(* Logix 5000 AddOnInstructionDefinition export HI6200_Faceplate_IT_AOI; software revision 30.00 *)

ADD_ON_INSTRUCTION HI6200_Faceplate_IT_AOI   (* revision 1.1, vendor Hardy Process Solutions *)
// HMI AOI for the Integrated Technician data.
VAR_IN_OUT
   Inp_hi6200 : _0102:Hardy6200Series_F6857DC7:I:0; {required}
   Out_hi6200 : _0102:Hardy6200Series_52E4DDE0:O:0; {required}
END_VAR
VAR_INPUT
   IT_Status : DINT;   // Integrated Technician status indication
   pm_4990 : REAL;   // WT ch 0
   pm_4991 : REAL;   // Wt ch 1
   pm_4992 : REAL;   // WT ch 2
   pm_4993 : REAL;   // WT ch 3
   pm_4994 : REAL;   // WT ch 4
   pm_4995 : REAL;   // WT ch 5
   pm_4996 : REAL;   // WT ch 6
   pm_4997 : REAL;   // WT ch 7
   pm_49A0 : REAL;   // mv/v ch 0
   pm_49A1 : REAL;   // mv/v ch 1
   pm_49A2 : REAL;   // mv/v ch 2
   pm_49A3 : REAL;   // mv/v ch 3
   pm_49A8 : REAL;   // mv/v ref 1
   pm_49A4 : REAL;   // mv/v ch 4
   pm_49A5 : REAL;   // mv/v ch 5
   pm_49A6 : REAL;   // mv/v ch 6
   pm_49A7 : REAL;   // mv/v ch 7
   pm_49A9 : REAL;   // mv/v ref 2
   pm_49B0 : REAL;   // RAW VAR ch 0
   pm_49B1 : REAL;   // RAW VAR ch 1
   pm_49B2 : REAL;   // RAW VAR ch 2
   pm_49B3 : REAL;   // RAW VAR ch 3
   pm_49B8 : REAL;   // RAW VAR ref 1
   pm_49B4 : REAL;   // RAW VAR ch 4
   pm_49B5 : REAL;   // RAW VAR ch 5
   pm_49B6 : REAL;   // RAW VAR ch 6
   pm_49B7 : REAL;   // RAW VAR ch 7
   pm_49B9 : REAL;   // RAW VAR ref 2
   pm_49C0 : REAL;   // WAVERSAVER VAR ch 0
   pm_49C1 : REAL;   // WAVERSAVER VAR ch 1
   pm_49C2 : REAL;   // WAVERSAVER VAR ch 2
   pm_49C3 : REAL;   // WAVERSAVER VAR ch 3
   pm_49C8 : REAL;   // WAVERSAVER VAR ref 1
   pm_49C4 : REAL;   // WAVERSAVER VAR ch 4
   pm_49C5 : REAL;   // WAVERSAVER VAR ch 5
   pm_49C6 : REAL;   // WAVERSAVER VAR ch 6
   pm_49C7 : REAL;   // WAVERSAVER VAR ch 7
   pm_49C9 : REAL;   // WAVERSAVER VAR ref 2
   pm_49D0 : DINT;   // RAW VAR results ch 0
   pm_49D1 : DINT;   // RAW VAR results ch 1
   pm_49D2 : DINT;   // RAW VAR results ch 2
   pm_49D3 : DINT;   // RAW VAR results ch 3
   pm_49D8 : DINT;   // RAW VAR results ref 1
   pm_49D4 : DINT;   // RAW VAR results ch 4
   pm_49D5 : DINT;   // RAW VAR results ch 5
   pm_49D6 : DINT;   // RAW VAR results ch 6
   pm_49D7 : DINT;   // RAW VAR results ch 7
   pm_49D9 : DINT;   // RAW VAR results ref 2
   pm_49E0 : DINT;   // WAVERSAVER VAR results ch 0
   pm_49E1 : DINT;   // WAVERSAVER VAR results ch 1
   pm_49E2 : DINT;   // WAVERSAVER VAR results ch 2
   pm_49E3 : DINT;   // WAVERSAVER VAR results ch 3
   pm_49E8 : DINT;   // WAVERSAVER VAR results ref 1
   pm_49E4 : DINT;   // WAVERSAVER VAR results ch 4
   pm_49E5 : DINT;   // WAVERSAVER VAR results ch 5
   pm_49E6 : DINT;   // WAVERSAVER VAR results ch 6
   pm_49E7 : DINT;   // WAVERSAVER VAR results ch 7
   pm_49E9 : DINT;   // WAVERSAVER VAR results ref 2
   rd_rtz : INT;   // return to zero status
   pm_49F0 : DINT;   // RTZ ch 0
   pm_49F1 : DINT;   // RTZ ch 1
   pm_49F2 : DINT;   // RTZ ch 2
   pm_49F3 : DINT;   // RTZ ch 3
   pm_49F4 : DINT;   // RTZ ch 4
   pm_49F5 : DINT;   // RTZ ch 5
   pm_49F6 : DINT;   // RTZ ch 6
   pm_49F7 : DINT;   // RTZ ch 7
   pm_498C : DINT;   // RTZ combined
   IT_button : INT;   // IT cmd from faceplate
        .0   // IT cmd from faceplate
   pm_4881 : DINT;   // Number IT jboxes
   pm_4103 : DINT;   // Number C2 sensors
   pm_498D : DINT;   // num sensors jbox 1
   pm_498E : DINT;   // num sensors jbox 2
   IT_reduce_button : INT;   // IT reduced cmd from faceplate
        .0   // IT reduced cmd from faceplate
   IT_running_status : DINT;   // running/status indication
END_VAR
VAR
   rd_IT_wt : INT; {access None}   // Trigger to check weights
   rd_mVV : INT; {access None}   // trigger to read mv/v
   rd_raw_var : INT; {access None}   // trigger to read raw variation
   rd_ws_var : INT; {access None}   // trigger to read WAVERSAVER variation
   rd_raw_rst : INT; {access None}   // trigger to read raw variation results
   rd_ws_rst : INT; {access None}   // trigger to read WAVERSAVER results
   IT_request : INT; {access None}   // type 1=standard 2=reduced
   IT_cmd : INT;   // trigger to run IT test
   wr_jbox_2 : BOOL; {access None}   // Process control bit
   two_jbox : BOOL; {access None}   // two IT j-box indication
   cmd_IT : DINT; {access None}   // holding register for command to be run
   IT_complete : BOOL; {access None}   // process status bit
   IT_failed : BOOL; {access None}   // process status bit
   write_box1_lc_cnt : BOOL; {access None}   // Process control bit
   write_box2_lc_cnt : BOOL; {access None}   // Process control bit
   c2_dev_notmatch : BOOL; {access None}   // status indication bit
   total_sensors : DINT; {access None}   // total sensors indication
   rd_jbox_2_too : BOOL; {access None}   // Process control bit
   delay_check2 : TIMER := (PRE := 1000); {access None}   // time delay to copy value
   delay_check1 : TIMER := (PRE := 1000); {access None}   // time delay to copy value
   read_delay_1 : TIMER := (PRE := 200); {access None}   // time delay to copy value
   delay_clear : TIMER := (PRE := 1000); {access None}   // time delay to copy value
   read_delay_2 : TIMER := (PRE := 200); {access None}   // time delay to copy value
   read_delay_3 : TIMER := (PRE := 200); {access None}   // time delay to copy value
   read_delay_4 : TIMER := (PRE := 200); {access None}   // time delay to copy value
   read_delay_5 : TIMER := (PRE := 200); {access None}   // time delay to copy value
   read_delay_6 : TIMER := (PRE := 200); {access None}   // time delay to copy value
   read_delay_7 : TIMER := (PRE := 200); {access None}   // time delay to copy value
   read_delay_8 : TIMER := (PRE := 200); {access None}   // time delay to copy value
   read_delay_9 : TIMER := (PRE := 200); {access None}   // time delay to copy value
   read_delay_10 : TIMER := (PRE := 200); {access None}   // time delay to copy value
   read_delay_11 : TIMER := (PRE := 200); {access None}   // time delay to copy value
   read_delay_12 : TIMER := (PRE := 200); {access None}   // time delay to copy value
   read_delay_13 : TIMER := (PRE := 200); {access None}   // time delay to copy value
   read_delay_14 : TIMER := (PRE := 200); {access None}   // time delay to copy value
   read_delay_15 : TIMER := (PRE := 200); {access None}   // time delay to copy value
   read_delay_16 : TIMER := (PRE := 200); {access None}   // time delay to copy value
   read_delay_17 : TIMER := (PRE := 200); {access None}   // time delay to copy value
   read_delay_18 : TIMER := (PRE := 200); {access None}   // time delay to copy value
   read_delay_19 : TIMER := (PRE := 200); {access None}   // time delay to copy value
   read_delay_20 : TIMER := (PRE := 200); {access None}   // time delay to copy value
   read_delay_21 : TIMER := (PRE := 200); {access None}   // time delay to copy value
   read_delay_22 : TIMER := (PRE := 200); {access None}   // time delay to copy value
   read_delay_23 : TIMER := (PRE := 200); {access None}   // time delay to copy value
   read_delay_24 : TIMER := (PRE := 200); {access None}   // time delay to copy value
   read_delay_25 : TIMER := (PRE := 200); {access None}   // time delay to copy value
   read_delay_26 : TIMER := (PRE := 200); {access None}   // time delay to copy value
   read_delay_27 : TIMER := (PRE := 200); {access None}   // time delay to copy value
   read_delay_28 : TIMER := (PRE := 200); {access None}   // time delay to copy value
   read_delay_29 : TIMER := (PRE := 200); {access None}   // time delay to copy value
   read_delay_30 : TIMER := (PRE := 200); {access None}   // time delay to copy value
   read_delay_31 : TIMER := (PRE := 200); {access None}   // time delay to copy value
   read_delay_32 : TIMER := (PRE := 200); {access None}   // time delay to copy value
   read_delay_33 : TIMER := (PRE := 200); {access None}   // time delay to copy value
   read_delay_34 : TIMER := (PRE := 200); {access None}   // time delay to copy value
   read_delay_35 : TIMER := (PRE := 200); {access None}   // time delay to copy value
   read_delay_36 : TIMER := (PRE := 200); {access None}   // time delay to copy value
   read_delay_37 : TIMER := (PRE := 200); {access None}   // time delay to copy value
   read_delay_38 : TIMER := (PRE := 200); {access None}   // time delay to copy value
   read_delay_39 : TIMER := (PRE := 200); {access None}   // time delay to copy value
   read_delay_40 : TIMER := (PRE := 200); {access None}   // time delay to copy value
   read_delay_41 : TIMER := (PRE := 200); {access None}   // time delay to copy value
   read_delay_42 : TIMER := (PRE := 200); {access None}   // time delay to copy value
   read_delay_43 : TIMER := (PRE := 200); {access None}   // time delay to copy value
   read_delay_44 : TIMER := (PRE := 200); {access None}   // time delay to copy value
   read_delay_45 : TIMER := (PRE := 200); {access None}   // time delay to copy value
   read_delay_46 : TIMER := (PRE := 200); {access None}   // time delay to copy value
   read_delay_47 : TIMER := (PRE := 200); {access None}   // time delay to copy value
   read_delay_48 : TIMER := (PRE := 200); {access None}   // time delay to copy value
   read_delay_49 : TIMER := (PRE := 200); {access None}   // time delay to copy value
   read_delay_50 : TIMER := (PRE := 200); {access None}   // time delay to copy value
   read_delay_51 : TIMER := (PRE := 200); {access None}   // time delay to copy value
   read_delay_52 : TIMER := (PRE := 200); {access None}   // time delay to copy value
   read_delay_53 : TIMER := (PRE := 200); {access None}   // time delay to copy value
   read_delay_54 : TIMER := (PRE := 200); {access None}   // time delay to copy value
   read_delay_55 : TIMER := (PRE := 200); {access None}   // time delay to copy value
   read_delay_56 : TIMER := (PRE := 200); {access None}   // time delay to copy value
   read_delay_57 : TIMER := (PRE := 200); {access None}   // time delay to copy value
   read_delay_58 : TIMER := (PRE := 200); {access None}   // time delay to copy value
   read_delay_59 : TIMER := (PRE := 200); {access None}   // time delay to copy value
   read_delay_60 : TIMER := (PRE := 200); {access None}   // time delay to copy value
   read_delay_61 : TIMER := (PRE := 200); {access None}   // time delay to copy value
   read_delay_62 : TIMER := (PRE := 200); {access None}   // time delay to copy value
   read_delay_63 : TIMER := (PRE := 200); {access None}   // time delay to copy value
   read_delay_64 : TIMER := (PRE := 200); {access None}   // time delay to copy value
   read_delay_65 : TIMER := (PRE := 200); {access None}   // time delay to copy value
   read_delay_66 : TIMER := (PRE := 200); {access None}   // time delay to copy value
   read_delay_67 : TIMER := (PRE := 200); {access None}   // time delay to copy value
   type_IT_cmd : BOOL; {access None}   // process control bit
   run_IT_test : BOOL; {access None}   // Process control bit
   run_C2_search : BOOL; {access None}   // Process control bit
   rd_num_sensors : BOOL; {access None}   // process control bit
   rd_num_j_boxes : BOOL; {access None}   // process control bit
   one_jbox : BOOL; {access None}   // One IT j-box found indication
   no_it_jbox : BOOL; {access None}   // no IT j-box indication
   jbox_check : BOOL; {access None}   // j-box check process bit
   clear_status : BOOL; {access None}   // process control bit
   c2_search_2 : BOOL; {access None}   // process control bit
   c2_search : BOOL; {access None}   // process control bit
   Cmd_Status : DINT; {access Read Only}   // command status
END_VAR

ROUTINE Logic   (* ladder *)
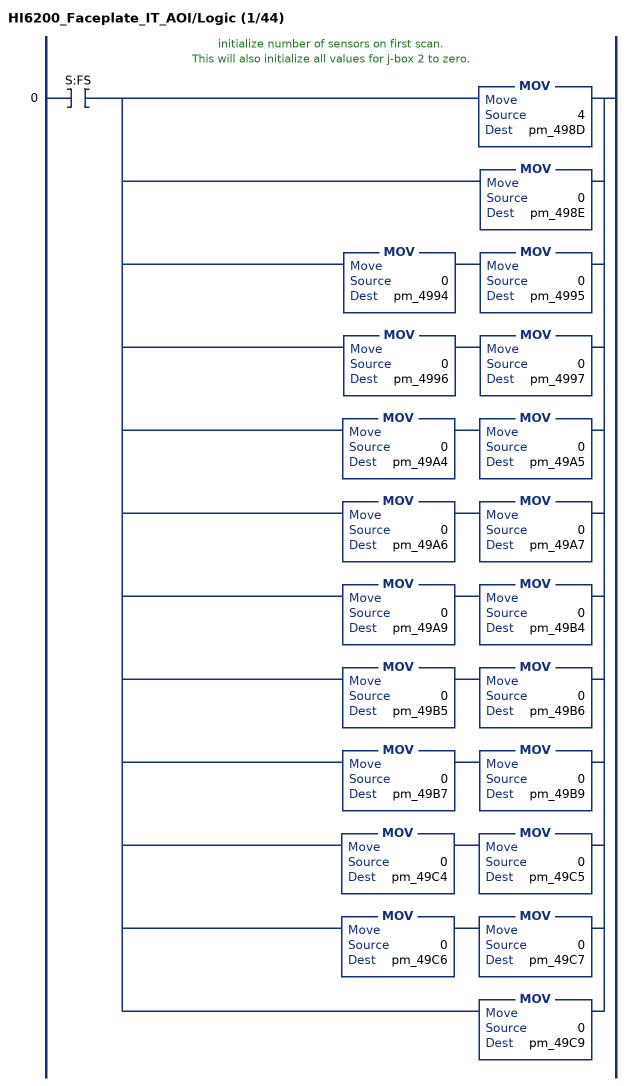
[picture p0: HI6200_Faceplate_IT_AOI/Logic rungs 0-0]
   // initialize number of sensors on first scan.
   // This will also initialize all values for j-box 2 to zero.
   0: XIC(S:FS)[MOV(4,pm_498D) ,MOV(0,pm_498E) ,MOV(0,pm_4994) MOV(0,pm_4995) ,MOV(0,pm_4996) MOV(0,pm_4997) ,MOV(0,pm_49A4) MOV(0,pm_49A5) ,MOV(0,pm_49A6) MOV(0,pm_49A7) ,MOV(0,pm_49A9) MOV(0,pm_49B4) ,MOV(0,pm_49B5) MOV(0,pm_49B6) ,MOV(0,pm_49B7) MOV(0,pm_49B9) ,MOV(0,pm_49C4) MOV(0,pm_49C5) ,MOV(0,pm_49C6) MOV(0,pm_49C7) ,MOV(0,pm_49C9) ];
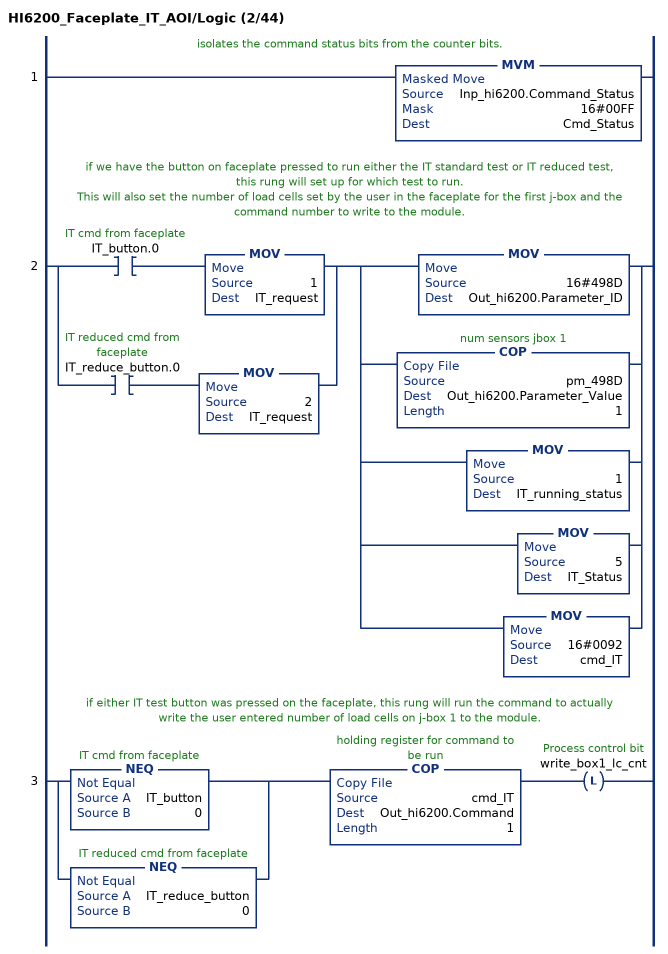
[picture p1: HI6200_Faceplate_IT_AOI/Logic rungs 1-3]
   // isolates the command status bits from the counter bits.
   1: MVM(Inp_hi6200.Command_Status,16#00FF,Cmd_Status);
   // if we have the button on faceplate pressed to run either the IT standard test or IT reduced test, this rung will set up for which test to run.
   // This will also set the number of load cells set by the user in the faceplate for the first j-box and the command number to write to the module.
   2: [XIC(IT_button.0) MOV(1,IT_request) ,XIC(IT_reduce_button.0) MOV(2,IT_request) ][MOV(16#498D,Out_hi6200.Parameter_ID) ,COP(pm_498D,Out_hi6200.Parameter_Value,1) ,MOV(1,IT_running_status) ,MOV(5,IT_Status) ,MOV(16#0092,cmd_IT) ];
   // if either IT test button was pressed on the faceplate, this rung will run the command to actually write the user entered number of load cells on j-box 1 to the module.
   3: [NEQ(IT_button,0) ,NEQ(IT_reduce_button,0) ]COP(cmd_IT,Out_hi6200.Command,1)OTL(write_box1_lc_cnt);
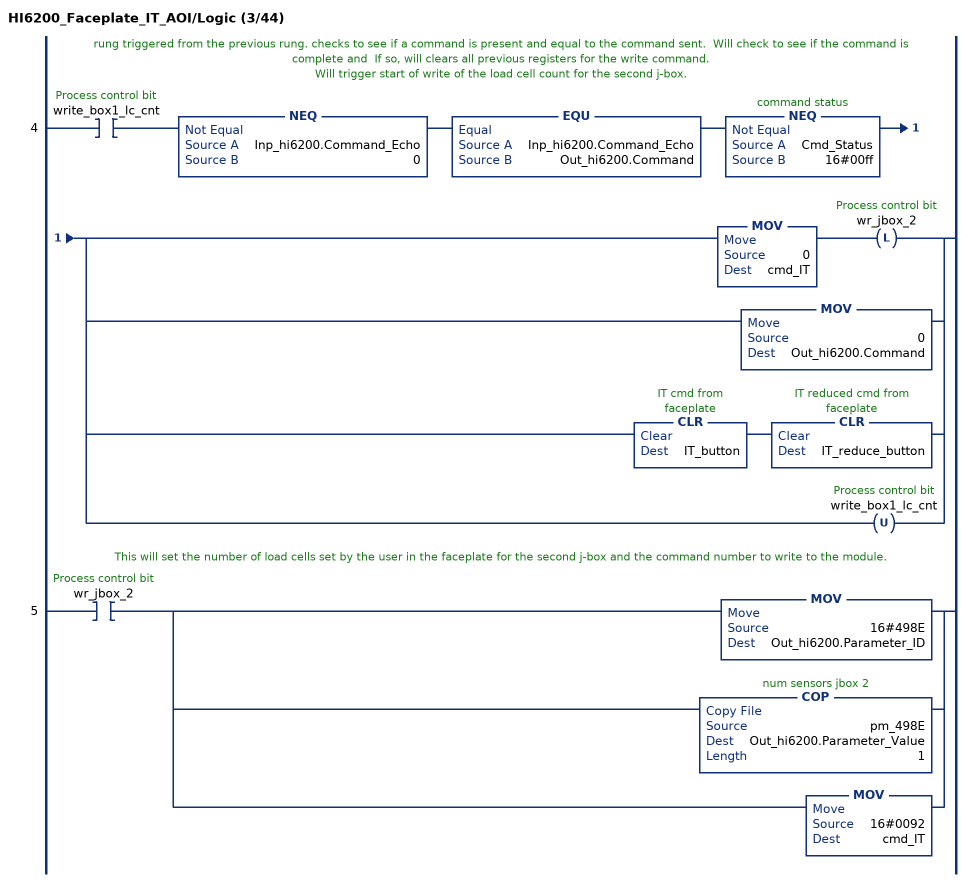
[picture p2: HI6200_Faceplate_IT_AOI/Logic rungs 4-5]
   // rung triggered from the previous rung. checks to see if a command is present and equal to the command sent.  Will check to see if the command is complete and  If so, will clears all previous registers for the write command.
   // Will trigger start of write of the load cell count for the second j-box.
   4: XIC(write_box1_lc_cnt)NEQ(Inp_hi6200.Command_Echo,0)EQU(Inp_hi6200.Command_Echo,Out_hi6200.Command)NEQ(Cmd_Status,16#00ff)[MOV(0,cmd_IT) OTL(wr_jbox_2) ,MOV(0,Out_hi6200.Command) ,CLR(IT_button) CLR(IT_reduce_button) ,OTU(write_box1_lc_cnt) ];
   // This will set the number of load cells set by the user in the faceplate for the second j-box and the command number to write to the module.
   5: XIC(wr_jbox_2)[MOV(16#498E,Out_hi6200.Parameter_ID) ,COP(pm_498E,Out_hi6200.Parameter_Value,1) ,MOV(16#0092,cmd_IT) ];
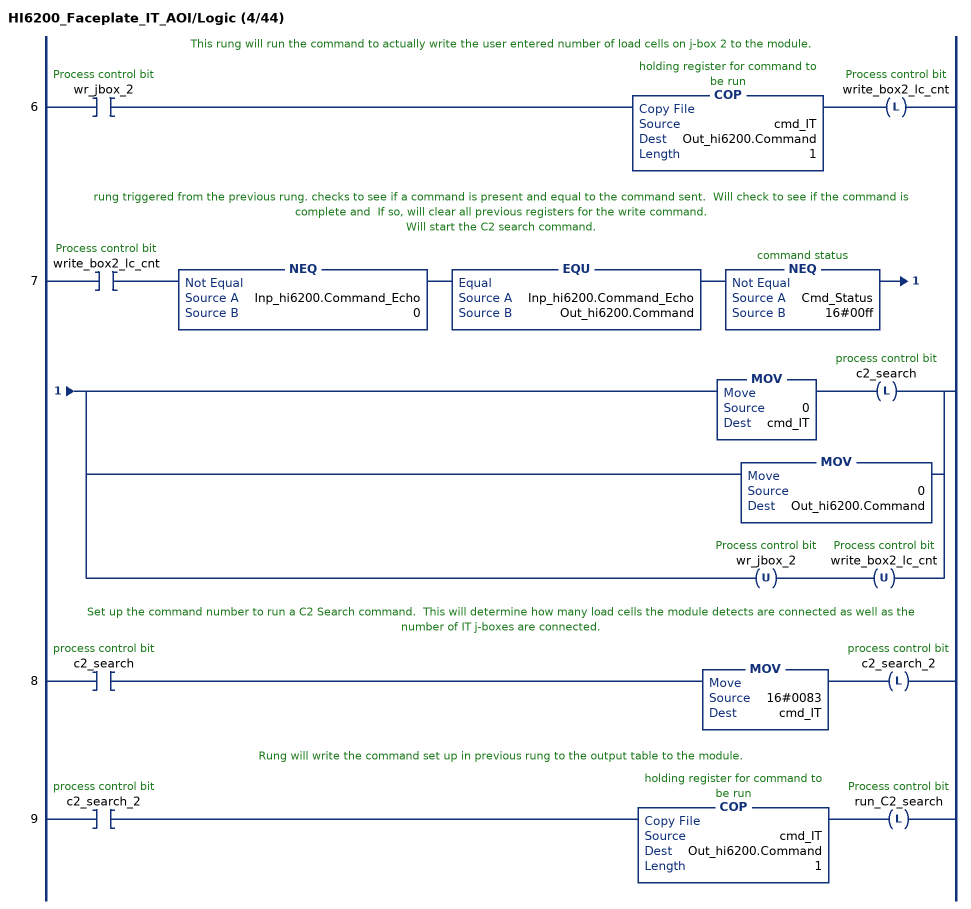
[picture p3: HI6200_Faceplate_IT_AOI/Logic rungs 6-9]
   // This rung will run the command to actually write the user entered number of load cells on j-box 2 to the module.
   6: XIC(wr_jbox_2)COP(cmd_IT,Out_hi6200.Command,1)OTL(write_box2_lc_cnt);
   // rung triggered from the previous rung. checks to see if a command is present and equal to the command sent.  Will check to see if the command is complete and  If so, will clear all previous registers for the write command.
   // Will start the C2 search command.
   7: XIC(write_box2_lc_cnt)NEQ(Inp_hi6200.Command_Echo,0)EQU(Inp_hi6200.Command_Echo,Out_hi6200.Command)NEQ(Cmd_Status,16#00ff)[MOV(0,cmd_IT) OTL(c2_search) ,MOV(0,Out_hi6200.Command) ,OTU(wr_jbox_2) OTU(write_box2_lc_cnt) ];
   // Set up the command number to run a C2 Search command.  This will determine how many load cells the module detects are connected as well as the number of IT j-boxes are connected.
   8: XIC(c2_search)MOV(16#0083,cmd_IT)OTL(c2_search_2);
   // Rung will write the command set up in previous rung to the output table to the module.
   9: XIC(c2_search_2)COP(cmd_IT,Out_hi6200.Command,1)OTL(run_C2_search);
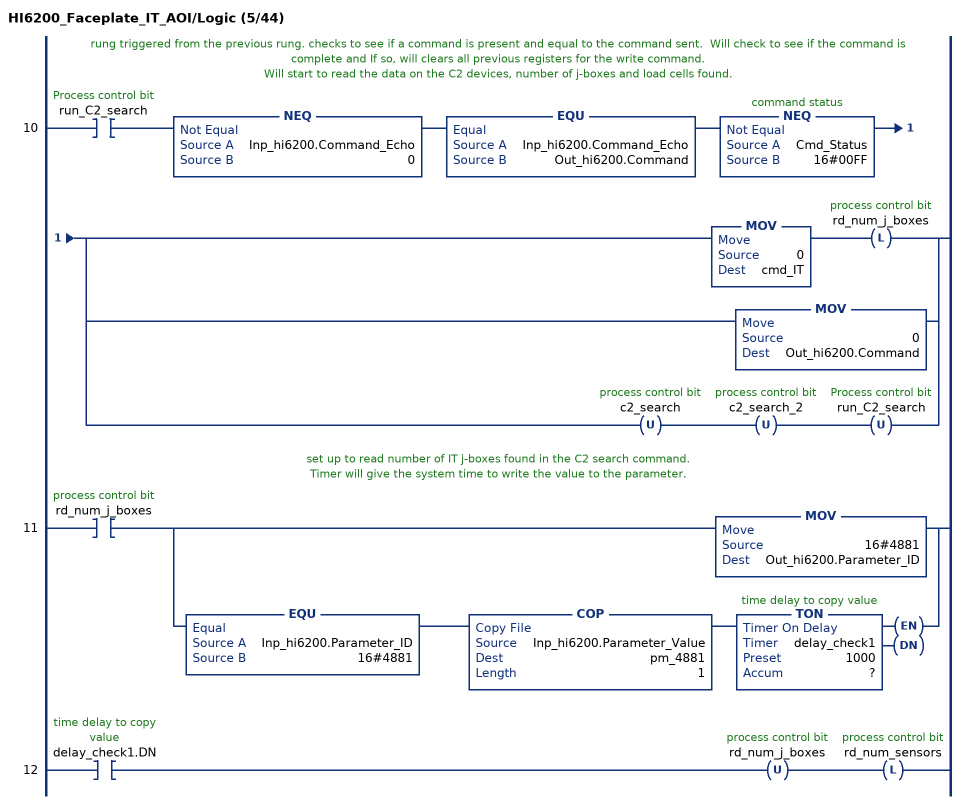
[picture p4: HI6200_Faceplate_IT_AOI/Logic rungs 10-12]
   // rung triggered from the previous rung. checks to see if a command is present and equal to the command sent.  Will check to see if the command is complete and If so, will clears all previous registers for the write command.
   // Will start to read the data on the C2 devices, number of j-boxes and load cells found.
   10: XIC(run_C2_search)NEQ(Inp_hi6200.Command_Echo,0)EQU(Inp_hi6200.Command_Echo,Out_hi6200.Command)NEQ(Cmd_Status,16#00FF)[MOV(0,cmd_IT) OTL(rd_num_j_boxes) ,MOV(0,Out_hi6200.Command) ,OTU(c2_search) OTU(c2_search_2) OTU(run_C2_search) ];
   // set up to read number of IT j-boxes found in the C2 search command.
   // Timer will give the system time to write the value to the parameter.
   11: XIC(rd_num_j_boxes)[MOV(16#4881,Out_hi6200.Parameter_ID) ,EQU(Inp_hi6200.Parameter_ID,16#4881) COP(Inp_hi6200.Parameter_Value,pm_4881,1) TON(delay_check1,?,?) ];
   12: XIC(delay_check1.DN)OTU(rd_num_j_boxes)OTL(rd_num_sensors);
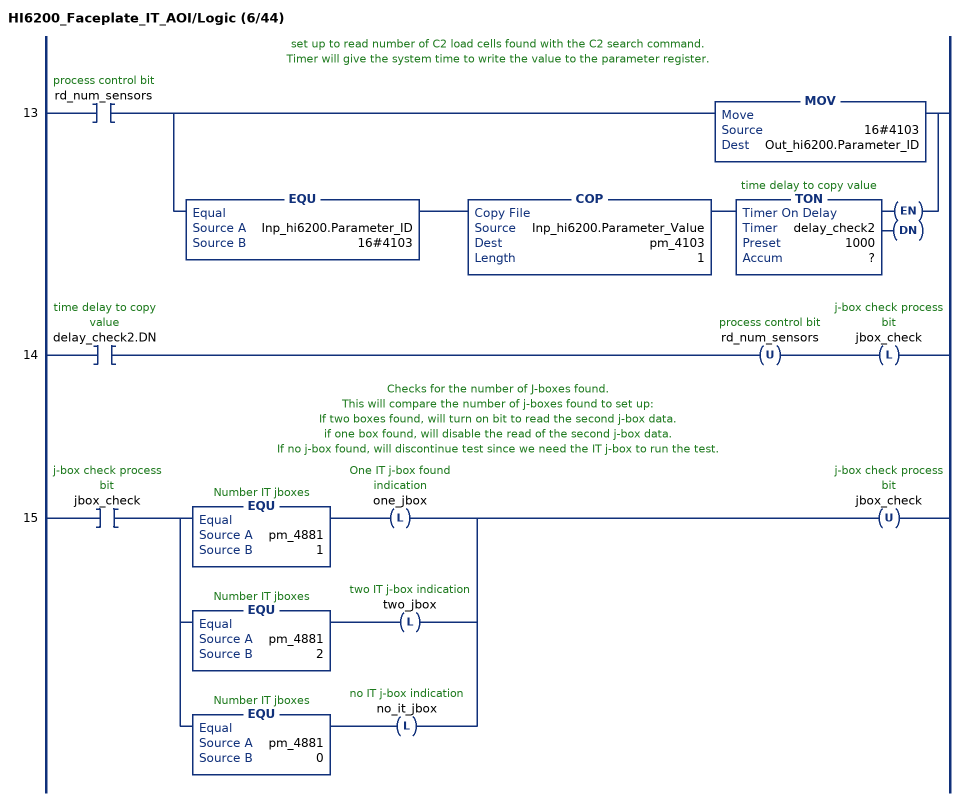
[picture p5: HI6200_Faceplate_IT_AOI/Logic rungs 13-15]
   // set up to read number of C2 load cells found with the C2 search command.
   // Timer will give the system time to write the value to the parameter register.
   13: XIC(rd_num_sensors)[MOV(16#4103,Out_hi6200.Parameter_ID) ,EQU(Inp_hi6200.Parameter_ID,16#4103) COP(Inp_hi6200.Parameter_Value,pm_4103,1) TON(delay_check2,?,?) ];
   14: XIC(delay_check2.DN)OTU(rd_num_sensors)OTL(jbox_check);
   // Checks for the number of J-boxes found.
   // This will compare the number of j-boxes found to set up:
   // If two boxes found, will turn on bit to read the second j-box data.
   // if one box found, will disable the read of the second j-box data.
   // If no j-box found, will discontinue test since we need the IT j-box to run the test.
   15: XIC(jbox_check)[EQU(pm_4881,1) OTL(one_jbox) ,EQU(pm_4881,2) OTL(two_jbox) ,EQU(pm_4881,0) OTL(no_it_jbox) ]OTU(jbox_check);
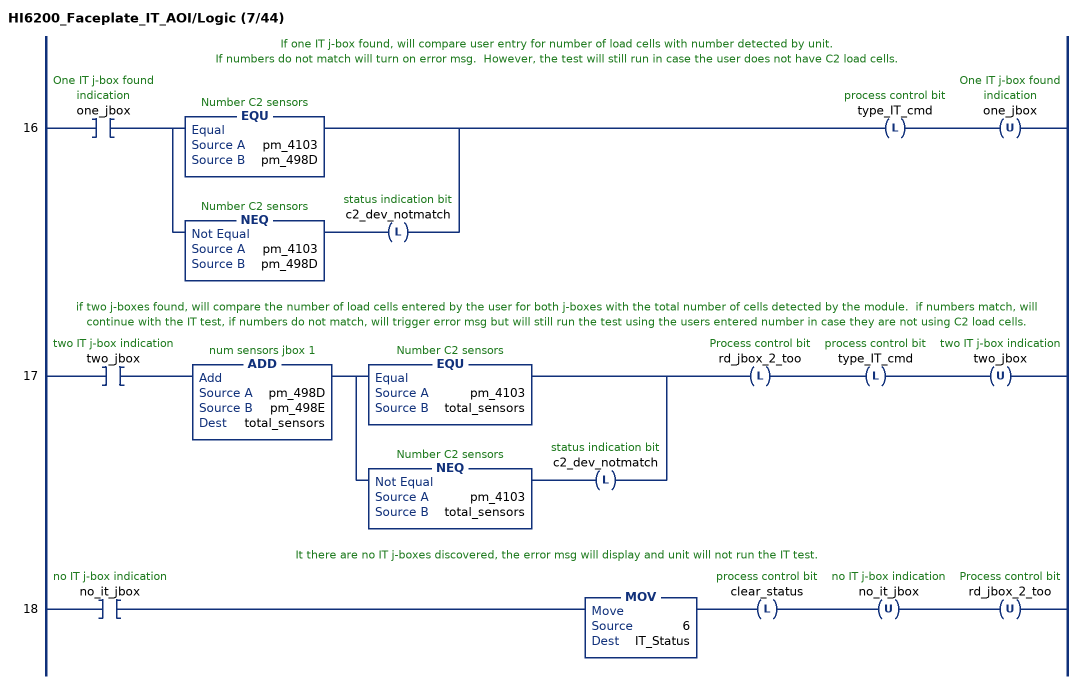
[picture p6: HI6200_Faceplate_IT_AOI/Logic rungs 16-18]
   // If one IT j-box found, will compare user entry for number of load cells with number detected by unit.
   // If numbers do not match will turn on error msg.  However, the test will still run in case the user does not have C2 load cells.
   16: XIC(one_jbox)[EQU(pm_4103,pm_498D) ,NEQ(pm_4103,pm_498D) OTL(c2_dev_notmatch) ]OTL(type_IT_cmd)OTU(one_jbox);
   // if two j-boxes found, will compare the number of load cells entered by the user for both j-boxes with the total number of cells detected by the module.  if numbers match, will continue with the IT test, if numbers do not match, will trigger error msg but will still run the test using the users entered number in case they are not using C2 load cells.
   17: XIC(two_jbox)ADD(pm_498D,pm_498E,total_sensors)[EQU(pm_4103,total_sensors) ,NEQ(pm_4103,total_sensors) OTL(c2_dev_notmatch) ]OTL(rd_jbox_2_too)OTL(type_IT_cmd)OTU(two_jbox);
   // It there are no IT j-boxes discovered, the error msg will display and unit will not run the IT test.
   18: XIC(no_it_jbox)MOV(6,IT_Status)OTL(clear_status)OTU(no_it_jbox)OTU(rd_jbox_2_too);
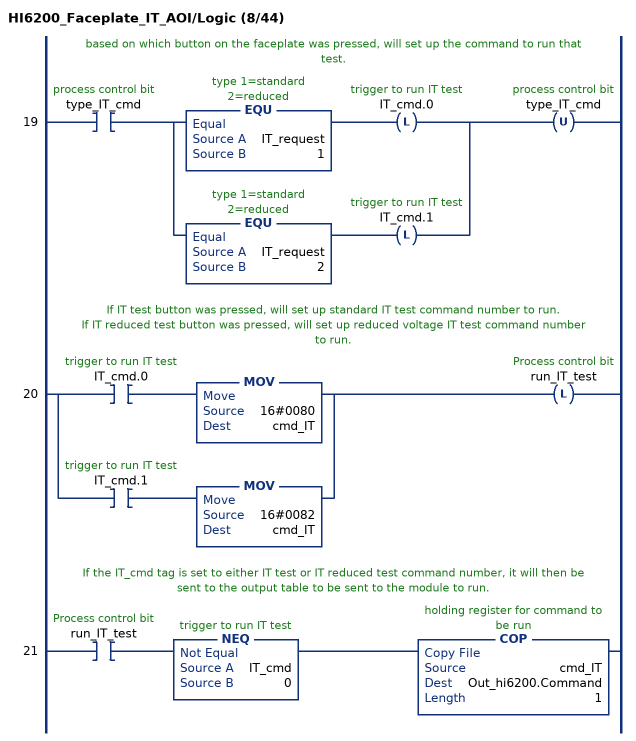
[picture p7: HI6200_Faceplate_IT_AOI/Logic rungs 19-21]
   // based on which button on the faceplate was pressed, will set up the command to run that test.
   19: XIC(type_IT_cmd)[EQU(IT_request,1) OTL(IT_cmd.0) ,EQU(IT_request,2) OTL(IT_cmd.1) ]OTU(type_IT_cmd);
   // If IT test button was pressed, will set up standard IT test command number to run.
   // If IT reduced test button was pressed, will set up reduced voltage IT test command number to run.
   20: [XIC(IT_cmd.0) MOV(16#0080,cmd_IT) ,XIC(IT_cmd.1) MOV(16#0082,cmd_IT) ]OTL(run_IT_test);
   // If the IT_cmd tag is set to either IT test or IT reduced test command number, it will then be sent to the output table to be sent to the module to run.
   21: XIC(run_IT_test)NEQ(IT_cmd,0)COP(cmd_IT,Out_hi6200.Command,1);
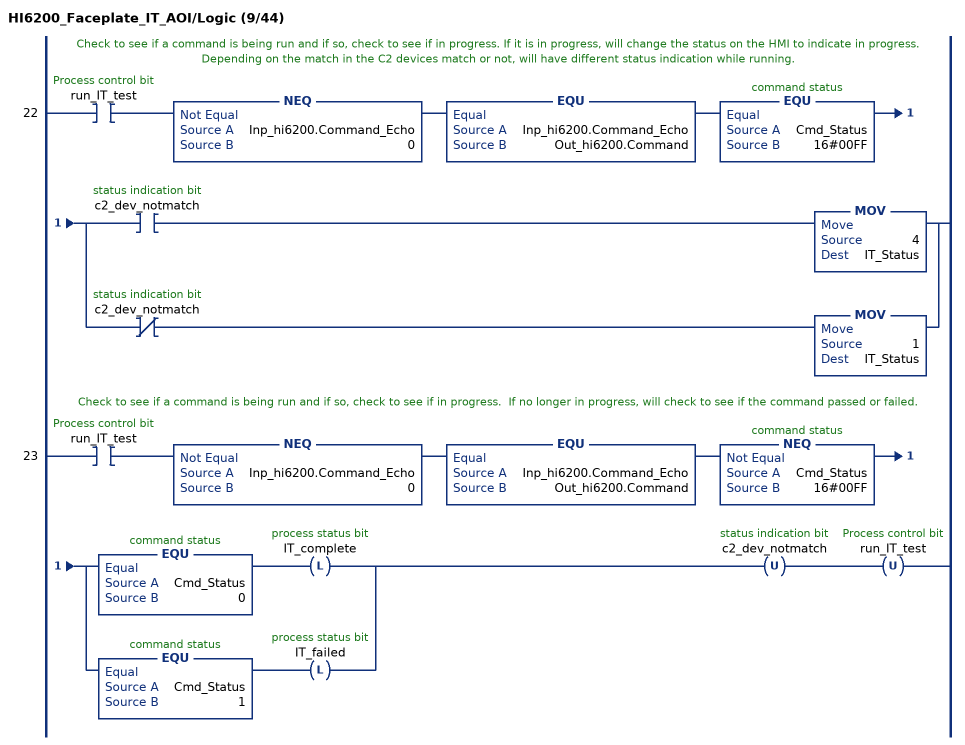
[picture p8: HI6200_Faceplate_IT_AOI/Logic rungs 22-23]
   // Check to see if a command is being run and if so, check to see if in progress. If it is in progress, will change the status on the HMI to indicate in progress.
   // Depending on the match in the C2 devices match or not, will have different status indication while running.
   22: XIC(run_IT_test)NEQ(Inp_hi6200.Command_Echo,0)EQU(Inp_hi6200.Command_Echo,Out_hi6200.Command)EQU(Cmd_Status,16#00FF)[XIC(c2_dev_notmatch) MOV(4,IT_Status) ,XIO(c2_dev_notmatch) MOV(1,IT_Status) ];
   // Check to see if a command is being run and if so, check to see if in progress.  If no longer in progress, will check to see if the command passed or failed.
   23: XIC(run_IT_test)NEQ(Inp_hi6200.Command_Echo,0)EQU(Inp_hi6200.Command_Echo,Out_hi6200.Command)NEQ(Cmd_Status,16#00FF)[EQU(Cmd_Status,0) OTL(IT_complete) ,EQU(Cmd_Status,1) OTL(IT_failed) ]OTU(c2_dev_notmatch)OTU(run_IT_test);
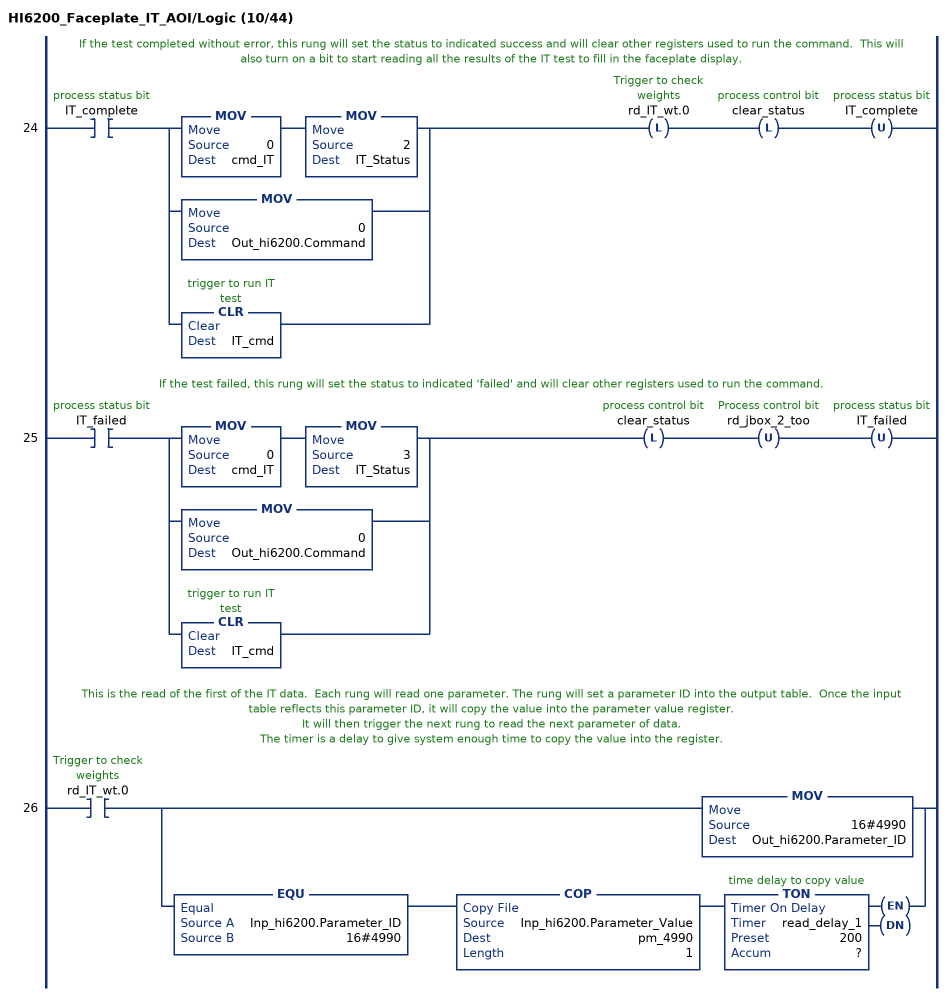
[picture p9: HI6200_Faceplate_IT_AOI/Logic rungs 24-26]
   // If the test completed without error, this rung will set the status to indicated success and will clear other registers used to run the command.  This will also turn on a bit to start reading all the results of the IT test to fill in the faceplate display.
   24: XIC(IT_complete)[MOV(0,cmd_IT) MOV(2,IT_Status) ,MOV(0,Out_hi6200.Command) ,CLR(IT_cmd) ]OTL(rd_IT_wt.0)OTL(clear_status)OTU(IT_complete);
   // If the test failed, this rung will set the status to indicated 'failed' and will clear other registers used to run the command.
   25: XIC(IT_failed)[MOV(0,cmd_IT) MOV(3,IT_Status) ,MOV(0,Out_hi6200.Command) ,CLR(IT_cmd) ]OTL(clear_status)OTU(rd_jbox_2_too)OTU(IT_failed);
   // This is the read of the first of the IT data.  Each rung will read one parameter. The rung will set a parameter ID into the output table.  Once the input table reflects this parameter ID, it will copy the value into the parameter value register.
   // It will then trigger the next rung to read the next parameter of data.
   // The timer is a delay to give system enough time to copy the value into the register.
   26: XIC(rd_IT_wt.0)[MOV(16#4990,Out_hi6200.Parameter_ID) ,EQU(Inp_hi6200.Parameter_ID,16#4990) COP(Inp_hi6200.Parameter_Value,pm_4990,1) TON(read_delay_1,?,?) ];
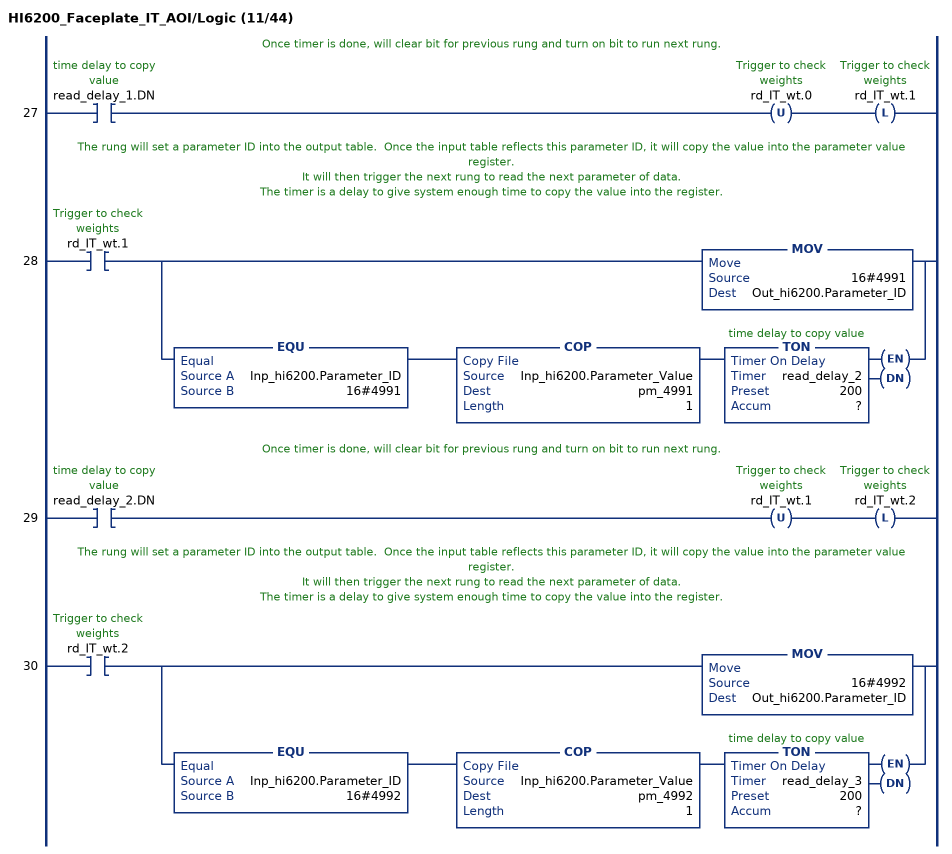
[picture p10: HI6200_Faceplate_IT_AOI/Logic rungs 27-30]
   // Once timer is done, will clear bit for previous rung and turn on bit to run next rung.
   27: XIC(read_delay_1.DN)OTU(rd_IT_wt.0)OTL(rd_IT_wt.1);
   // The rung will set a parameter ID into the output table.  Once the input table reflects this parameter ID, it will copy the value into the parameter value register.
   // It will then trigger the next rung to read the next parameter of data.
   // The timer is a delay to give system enough time to copy the value into the register.
   28: XIC(rd_IT_wt.1)[MOV(16#4991,Out_hi6200.Parameter_ID) ,EQU(Inp_hi6200.Parameter_ID,16#4991) COP(Inp_hi6200.Parameter_Value,pm_4991,1) TON(read_delay_2,?,?) ];
   // Once timer is done, will clear bit for previous rung and turn on bit to run next rung.
   29: XIC(read_delay_2.DN)OTU(rd_IT_wt.1)OTL(rd_IT_wt.2);
   // The rung will set a parameter ID into the output table.  Once the input table reflects this parameter ID, it will copy the value into the parameter value register.
   // It will then trigger the next rung to read the next parameter of data.
   // The timer is a delay to give system enough time to copy the value into the register.
   30: XIC(rd_IT_wt.2)[MOV(16#4992,Out_hi6200.Parameter_ID) ,EQU(Inp_hi6200.Parameter_ID,16#4992) COP(Inp_hi6200.Parameter_Value,pm_4992,1) TON(read_delay_3,?,?) ];
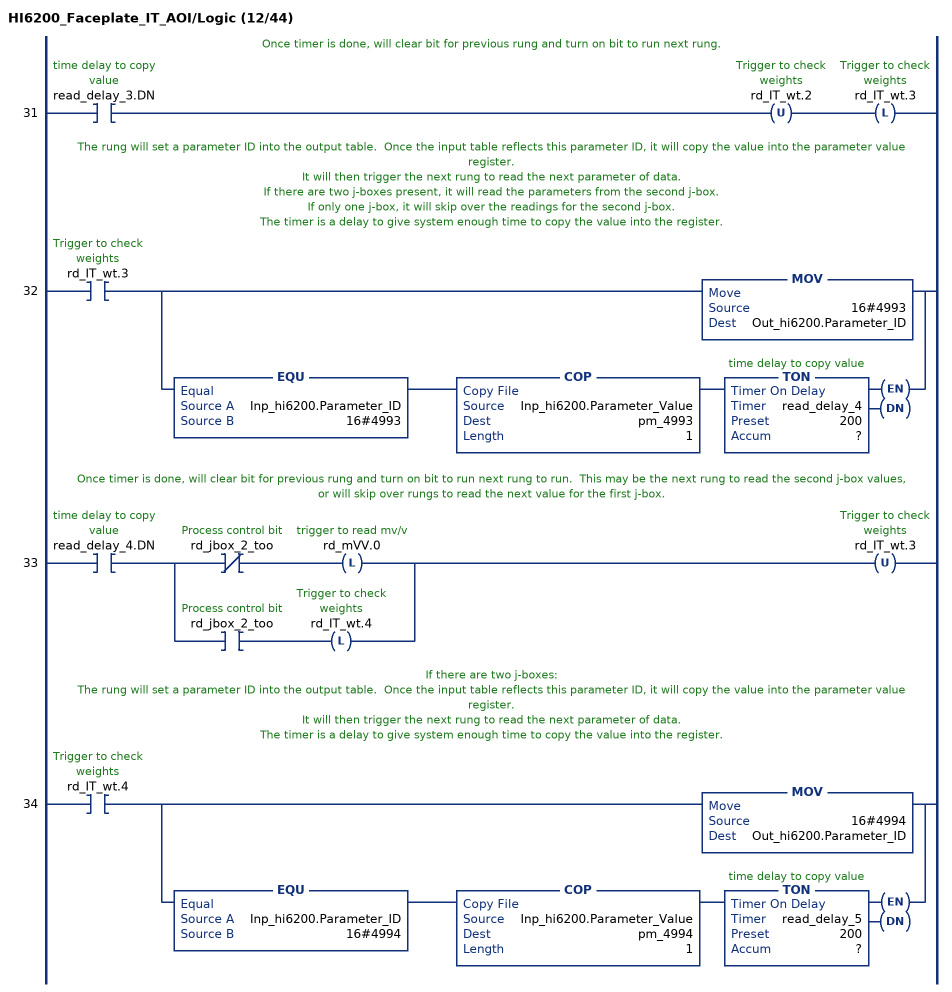
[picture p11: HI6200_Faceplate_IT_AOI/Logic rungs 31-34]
   // Once timer is done, will clear bit for previous rung and turn on bit to run next rung.
   31: XIC(read_delay_3.DN)OTU(rd_IT_wt.2)OTL(rd_IT_wt.3);
   // The rung will set a parameter ID into the output table.  Once the input table reflects this parameter ID, it will copy the value into the parameter value register.
   // It will then trigger the next rung to read the next parameter of data.
   // If there are two j-boxes present, it will read the parameters from the second j-box.
   // If only one j-box, it will skip over the readings for the second j-box.
   // The timer is a delay to give system enough time to copy the value into the register.
   32: XIC(rd_IT_wt.3)[MOV(16#4993,Out_hi6200.Parameter_ID) ,EQU(Inp_hi6200.Parameter_ID,16#4993) COP(Inp_hi6200.Parameter_Value,pm_4993,1) TON(read_delay_4,?,?) ];
   // Once timer is done, will clear bit for previous rung and turn on bit to run next rung to run.  This may be the next rung to read the second j-box values, or will skip over rungs to read the next value for the first j-box.
   33: XIC(read_delay_4.DN)[XIO(rd_jbox_2_too) OTL(rd_mVV.0) ,XIC(rd_jbox_2_too) OTL(rd_IT_wt.4) ]OTU(rd_IT_wt.3);
   // If there are two j-boxes:
   // The rung will set a parameter ID into the output table.  Once the input table reflects this parameter ID, it will copy the value into the parameter value register.
   // It will then trigger the next rung to read the next parameter of data.
   // The timer is a delay to give system enough time to copy the value into the register.
   34: XIC(rd_IT_wt.4)[MOV(16#4994,Out_hi6200.Parameter_ID) ,EQU(Inp_hi6200.Parameter_ID,16#4994) COP(Inp_hi6200.Parameter_Value,pm_4994,1) TON(read_delay_5,?,?) ];
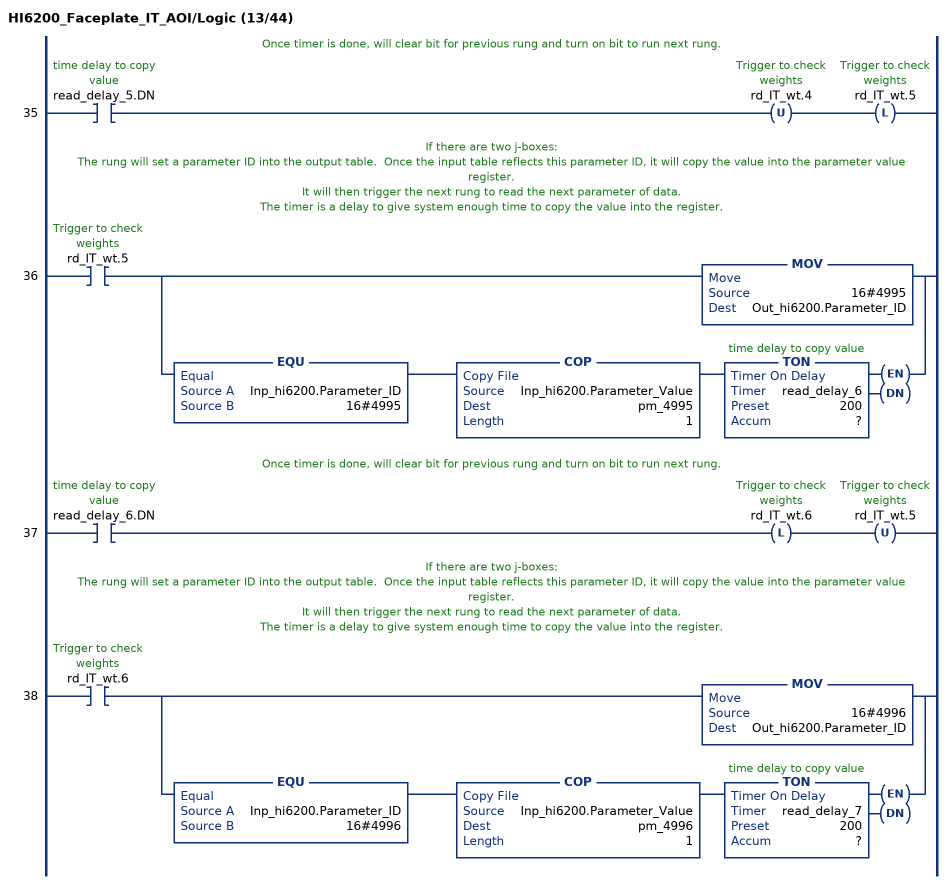
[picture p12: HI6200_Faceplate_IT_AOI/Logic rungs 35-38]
   // Once timer is done, will clear bit for previous rung and turn on bit to run next rung.
   35: XIC(read_delay_5.DN)OTU(rd_IT_wt.4)OTL(rd_IT_wt.5);
   // If there are two j-boxes:
   // The rung will set a parameter ID into the output table.  Once the input table reflects this parameter ID, it will copy the value into the parameter value register.
   // It will then trigger the next rung to read the next parameter of data.
   // The timer is a delay to give system enough time to copy the value into the register.
   36: XIC(rd_IT_wt.5)[MOV(16#4995,Out_hi6200.Parameter_ID) ,EQU(Inp_hi6200.Parameter_ID,16#4995) COP(Inp_hi6200.Parameter_Value,pm_4995,1) TON(read_delay_6,?,?) ];
   // Once timer is done, will clear bit for previous rung and turn on bit to run next rung.
   37: XIC(read_delay_6.DN)OTL(rd_IT_wt.6)OTU(rd_IT_wt.5);
   // If there are two j-boxes:
   // The rung will set a parameter ID into the output table.  Once the input table reflects this parameter ID, it will copy the value into the parameter value register.
   // It will then trigger the next rung to read the next parameter of data.
   // The timer is a delay to give system enough time to copy the value into the register.
   38: XIC(rd_IT_wt.6)[MOV(16#4996,Out_hi6200.Parameter_ID) ,EQU(Inp_hi6200.Parameter_ID,16#4996) COP(Inp_hi6200.Parameter_Value,pm_4996,1) TON(read_delay_7,?,?) ];
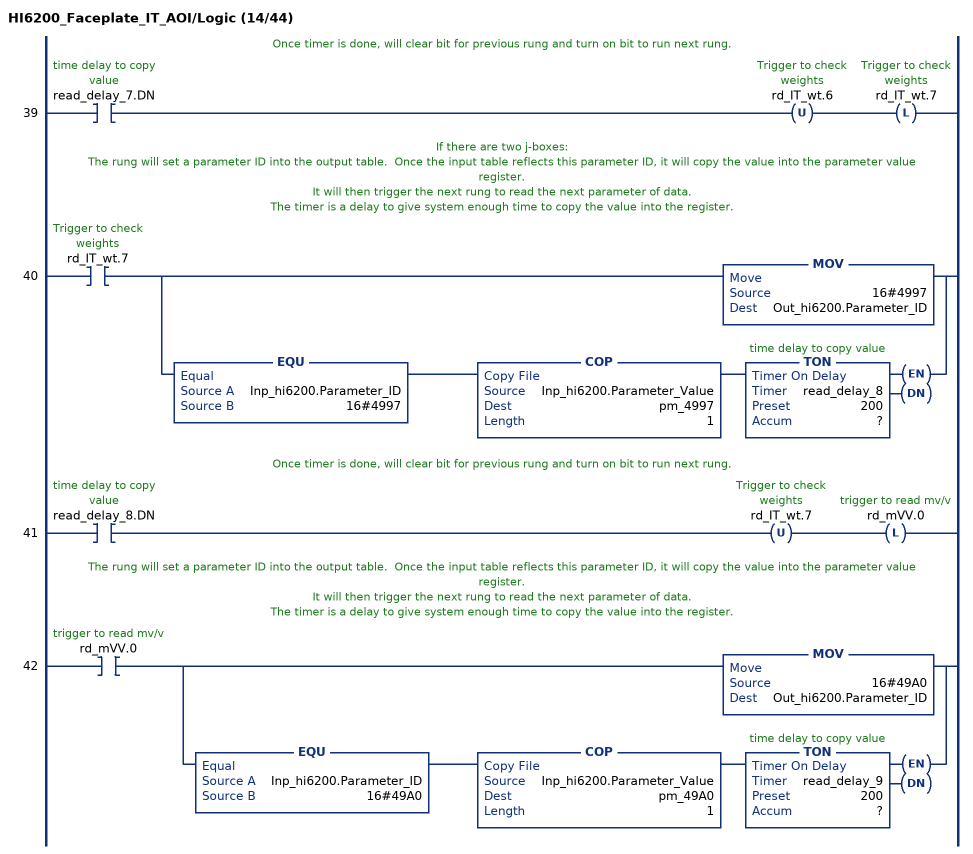
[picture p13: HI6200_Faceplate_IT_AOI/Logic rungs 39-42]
   // Once timer is done, will clear bit for previous rung and turn on bit to run next rung.
   39: XIC(read_delay_7.DN)OTU(rd_IT_wt.6)OTL(rd_IT_wt.7);
   // If there are two j-boxes:
   // The rung will set a parameter ID into the output table.  Once the input table reflects this parameter ID, it will copy the value into the parameter value register.
   // It will then trigger the next rung to read the next parameter of data.
   // The timer is a delay to give system enough time to copy the value into the register.
   40: XIC(rd_IT_wt.7)[MOV(16#4997,Out_hi6200.Parameter_ID) ,EQU(Inp_hi6200.Parameter_ID,16#4997) COP(Inp_hi6200.Parameter_Value,pm_4997,1) TON(read_delay_8,?,?) ];
   // Once timer is done, will clear bit for previous rung and turn on bit to run next rung.
   41: XIC(read_delay_8.DN)OTU(rd_IT_wt.7)OTL(rd_mVV.0);
   // The rung will set a parameter ID into the output table.  Once the input table reflects this parameter ID, it will copy the value into the parameter value register.
   // It will then trigger the next rung to read the next parameter of data.
   // The timer is a delay to give system enough time to copy the value into the register.
   42: XIC(rd_mVV.0)[MOV(16#49A0,Out_hi6200.Parameter_ID) ,EQU(Inp_hi6200.Parameter_ID,16#49A0) COP(Inp_hi6200.Parameter_Value,pm_49A0,1) TON(read_delay_9,?,?) ];
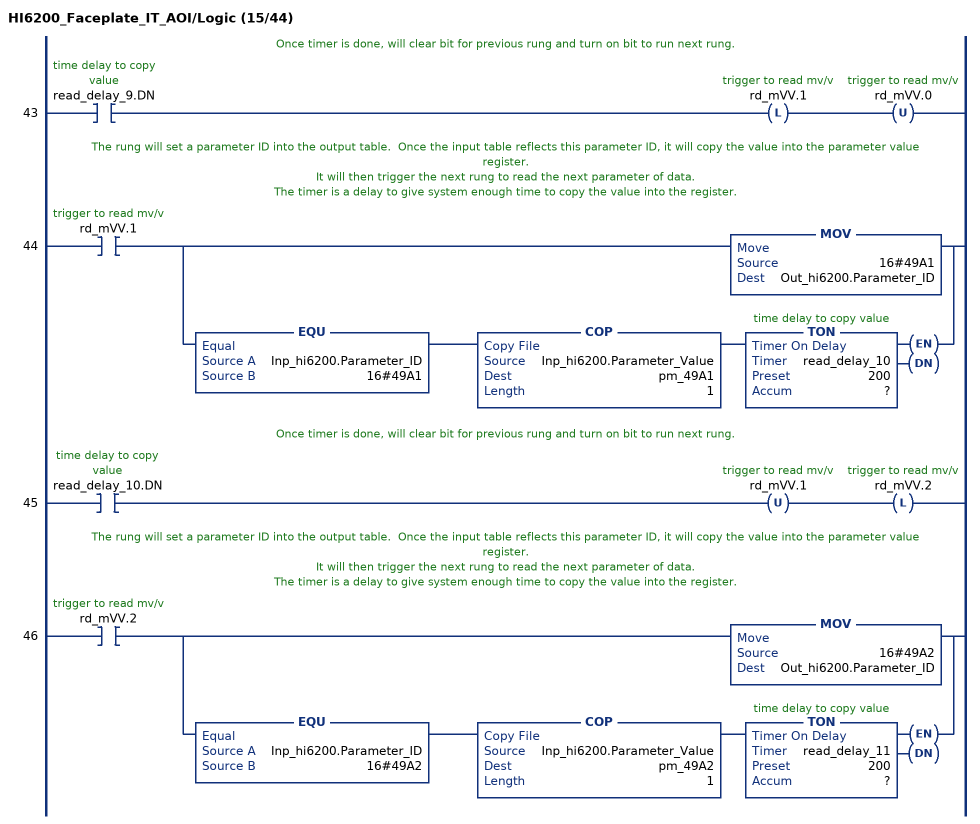
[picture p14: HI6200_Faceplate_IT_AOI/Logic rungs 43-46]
   // Once timer is done, will clear bit for previous rung and turn on bit to run next rung.
   43: XIC(read_delay_9.DN)OTL(rd_mVV.1)OTU(rd_mVV.0);
   // The rung will set a parameter ID into the output table.  Once the input table reflects this parameter ID, it will copy the value into the parameter value register.
   // It will then trigger the next rung to read the next parameter of data.
   // The timer is a delay to give system enough time to copy the value into the register.
   44: XIC(rd_mVV.1)[MOV(16#49A1,Out_hi6200.Parameter_ID) ,EQU(Inp_hi6200.Parameter_ID,16#49A1) COP(Inp_hi6200.Parameter_Value,pm_49A1,1) TON(read_delay_10,?,?) ];
   // Once timer is done, will clear bit for previous rung and turn on bit to run next rung.
   45: XIC(read_delay_10.DN)OTU(rd_mVV.1)OTL(rd_mVV.2);
   // The rung will set a parameter ID into the output table.  Once the input table reflects this parameter ID, it will copy the value into the parameter value register.
   // It will then trigger the next rung to read the next parameter of data.
   // The timer is a delay to give system enough time to copy the value into the register.
   46: XIC(rd_mVV.2)[MOV(16#49A2,Out_hi6200.Parameter_ID) ,EQU(Inp_hi6200.Parameter_ID,16#49A2) COP(Inp_hi6200.Parameter_Value,pm_49A2,1) TON(read_delay_11,?,?) ];
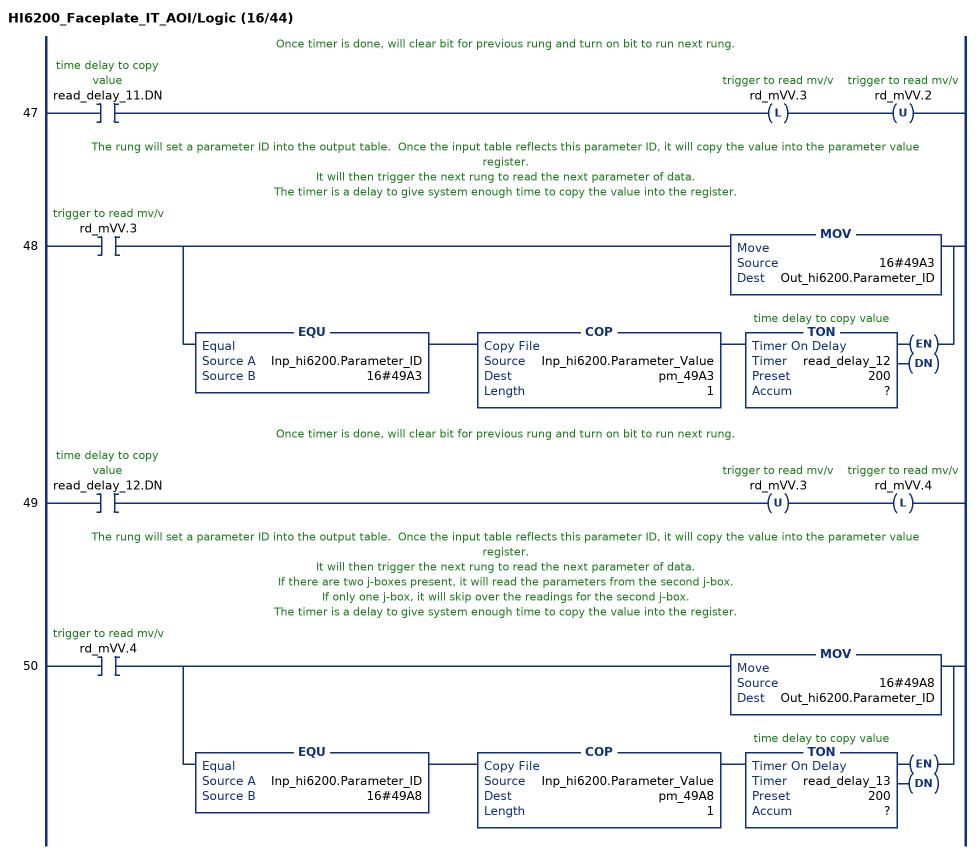
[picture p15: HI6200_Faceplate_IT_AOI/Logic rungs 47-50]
   // Once timer is done, will clear bit for previous rung and turn on bit to run next rung.
   47: XIC(read_delay_11.DN)OTL(rd_mVV.3)OTU(rd_mVV.2);
   // The rung will set a parameter ID into the output table.  Once the input table reflects this parameter ID, it will copy the value into the parameter value register.
   // It will then trigger the next rung to read the next parameter of data.
   // The timer is a delay to give system enough time to copy the value into the register.
   48: XIC(rd_mVV.3)[MOV(16#49A3,Out_hi6200.Parameter_ID) ,EQU(Inp_hi6200.Parameter_ID,16#49A3) COP(Inp_hi6200.Parameter_Value,pm_49A3,1) TON(read_delay_12,?,?) ];
   // Once timer is done, will clear bit for previous rung and turn on bit to run next rung.
   49: XIC(read_delay_12.DN)OTU(rd_mVV.3)OTL(rd_mVV.4);
   // The rung will set a parameter ID into the output table.  Once the input table reflects this parameter ID, it will copy the value into the parameter value register.
   // It will then trigger the next rung to read the next parameter of data.
   // If there are two j-boxes present, it will read the parameters from the second j-box.
   // If only one j-box, it will skip over the readings for the second j-box.
   // The timer is a delay to give system enough time to copy the value into the register.
   50: XIC(rd_mVV.4)[MOV(16#49A8,Out_hi6200.Parameter_ID) ,EQU(Inp_hi6200.Parameter_ID,16#49A8) COP(Inp_hi6200.Parameter_Value,pm_49A8,1) TON(read_delay_13,?,?) ];
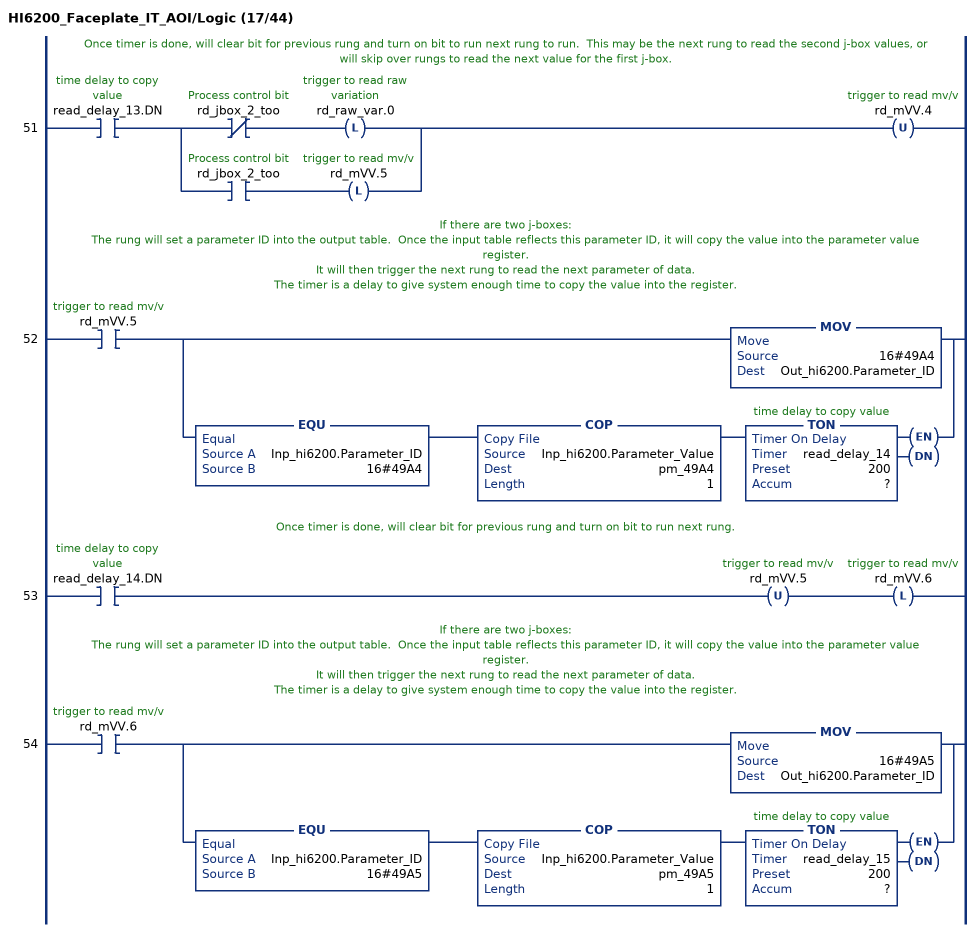
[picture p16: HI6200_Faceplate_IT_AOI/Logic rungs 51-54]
   // Once timer is done, will clear bit for previous rung and turn on bit to run next rung to run.  This may be the next rung to read the second j-box values, or will skip over rungs to read the next value for the first j-box.
   51: XIC(read_delay_13.DN)[XIO(rd_jbox_2_too) OTL(rd_raw_var.0) ,XIC(rd_jbox_2_too) OTL(rd_mVV.5) ]OTU(rd_mVV.4);
   // If there are two j-boxes:
   // The rung will set a parameter ID into the output table.  Once the input table reflects this parameter ID, it will copy the value into the parameter value register.
   // It will then trigger the next rung to read the next parameter of data.
   // The timer is a delay to give system enough time to copy the value into the register.
   52: XIC(rd_mVV.5)[MOV(16#49A4,Out_hi6200.Parameter_ID) ,EQU(Inp_hi6200.Parameter_ID,16#49A4) COP(Inp_hi6200.Parameter_Value,pm_49A4,1) TON(read_delay_14,?,?) ];
   // Once timer is done, will clear bit for previous rung and turn on bit to run next rung.
   53: XIC(read_delay_14.DN)OTU(rd_mVV.5)OTL(rd_mVV.6);
   // If there are two j-boxes:
   // The rung will set a parameter ID into the output table.  Once the input table reflects this parameter ID, it will copy the value into the parameter value register.
   // It will then trigger the next rung to read the next parameter of data.
   // The timer is a delay to give system enough time to copy the value into the register.
   54: XIC(rd_mVV.6)[MOV(16#49A5,Out_hi6200.Parameter_ID) ,EQU(Inp_hi6200.Parameter_ID,16#49A5) COP(Inp_hi6200.Parameter_Value,pm_49A5,1) TON(read_delay_15,?,?) ];
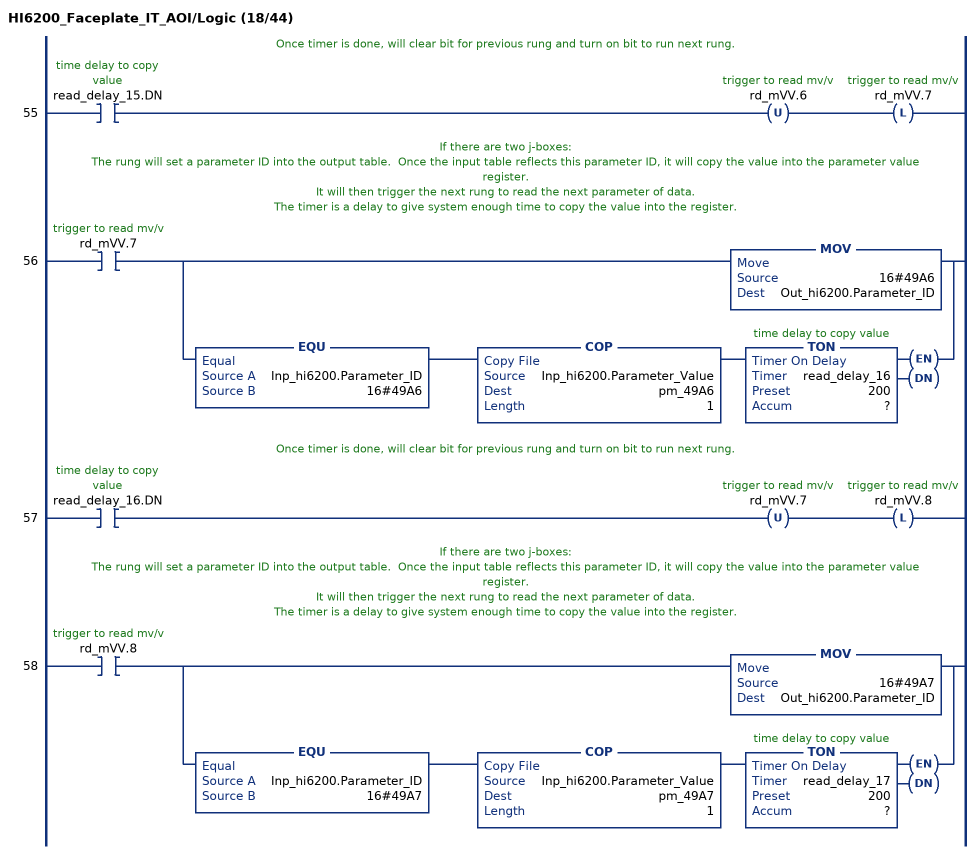
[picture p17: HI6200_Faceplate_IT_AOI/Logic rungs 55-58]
   // Once timer is done, will clear bit for previous rung and turn on bit to run next rung.
   55: XIC(read_delay_15.DN)OTU(rd_mVV.6)OTL(rd_mVV.7);
   // If there are two j-boxes:
   // The rung will set a parameter ID into the output table.  Once the input table reflects this parameter ID, it will copy the value into the parameter value register.
   // It will then trigger the next rung to read the next parameter of data.
   // The timer is a delay to give system enough time to copy the value into the register.
   56: XIC(rd_mVV.7)[MOV(16#49A6,Out_hi6200.Parameter_ID) ,EQU(Inp_hi6200.Parameter_ID,16#49A6) COP(Inp_hi6200.Parameter_Value,pm_49A6,1) TON(read_delay_16,?,?) ];
   // Once timer is done, will clear bit for previous rung and turn on bit to run next rung.
   57: XIC(read_delay_16.DN)OTU(rd_mVV.7)OTL(rd_mVV.8);
   // If there are two j-boxes:
   // The rung will set a parameter ID into the output table.  Once the input table reflects this parameter ID, it will copy the value into the parameter value register.
   // It will then trigger the next rung to read the next parameter of data.
   // The timer is a delay to give system enough time to copy the value into the register.
   58: XIC(rd_mVV.8)[MOV(16#49A7,Out_hi6200.Parameter_ID) ,EQU(Inp_hi6200.Parameter_ID,16#49A7) COP(Inp_hi6200.Parameter_Value,pm_49A7,1) TON(read_delay_17,?,?) ];
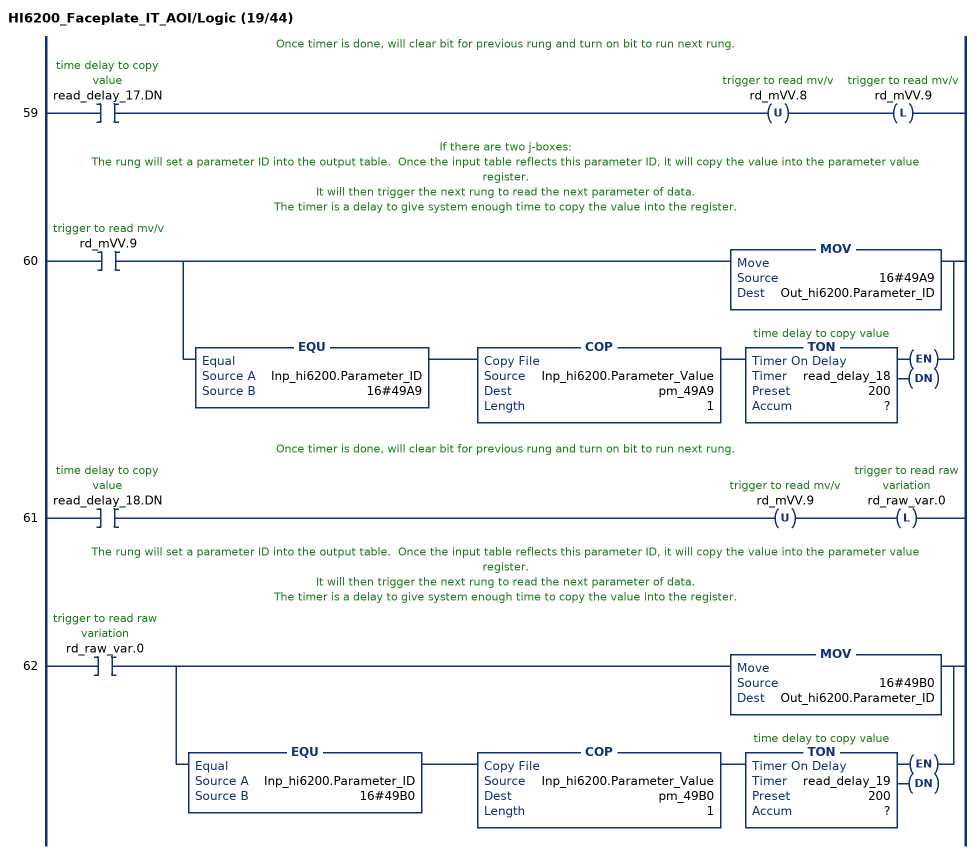
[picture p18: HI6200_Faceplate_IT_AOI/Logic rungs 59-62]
   // Once timer is done, will clear bit for previous rung and turn on bit to run next rung.
   59: XIC(read_delay_17.DN)OTU(rd_mVV.8)OTL(rd_mVV.9);
   // If there are two j-boxes:
   // The rung will set a parameter ID into the output table.  Once the input table reflects this parameter ID, it will copy the value into the parameter value register.
   // It will then trigger the next rung to read the next parameter of data.
   // The timer is a delay to give system enough time to copy the value into the register.
   60: XIC(rd_mVV.9)[MOV(16#49A9,Out_hi6200.Parameter_ID) ,EQU(Inp_hi6200.Parameter_ID,16#49A9) COP(Inp_hi6200.Parameter_Value,pm_49A9,1) TON(read_delay_18,?,?) ];
   // Once timer is done, will clear bit for previous rung and turn on bit to run next rung.
   61: XIC(read_delay_18.DN)OTU(rd_mVV.9)OTL(rd_raw_var.0);
   // The rung will set a parameter ID into the output table.  Once the input table reflects this parameter ID, it will copy the value into the parameter value register.
   // It will then trigger the next rung to read the next parameter of data.
   // The timer is a delay to give system enough time to copy the value into the register.
   62: XIC(rd_raw_var.0)[MOV(16#49B0,Out_hi6200.Parameter_ID) ,EQU(Inp_hi6200.Parameter_ID,16#49B0) COP(Inp_hi6200.Parameter_Value,pm_49B0,1) TON(read_delay_19,?,?) ];
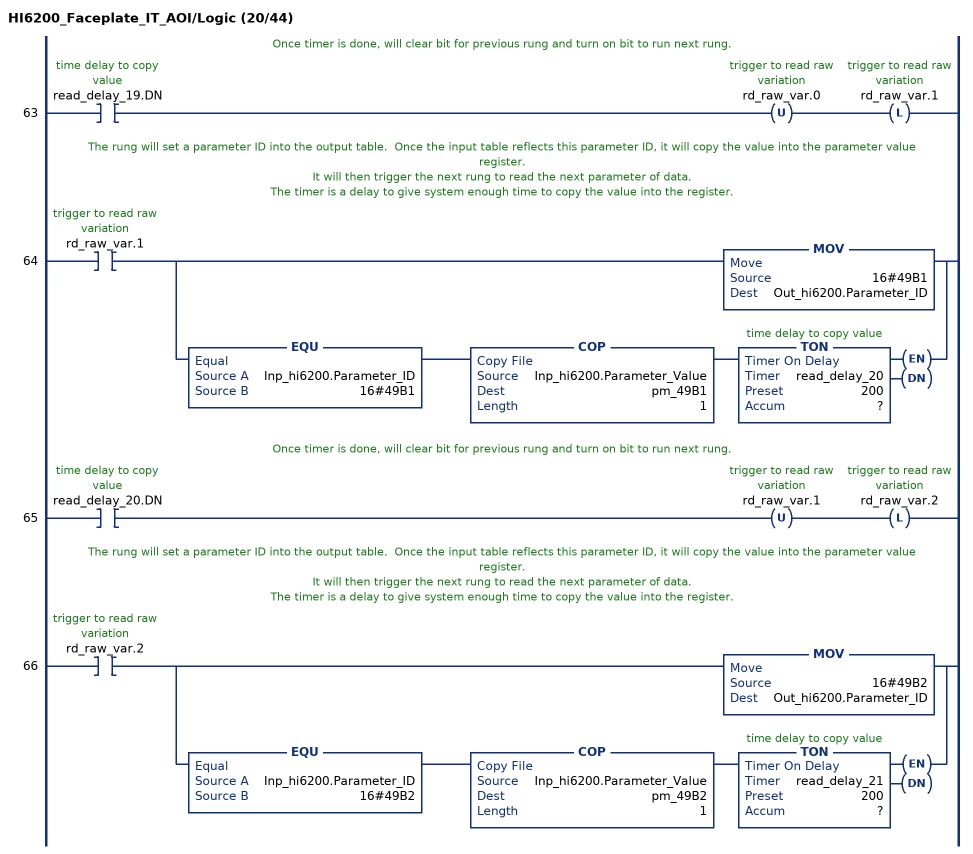
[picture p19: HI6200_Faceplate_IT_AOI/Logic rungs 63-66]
   // Once timer is done, will clear bit for previous rung and turn on bit to run next rung.
   63: XIC(read_delay_19.DN)OTU(rd_raw_var.0)OTL(rd_raw_var.1);
   // The rung will set a parameter ID into the output table.  Once the input table reflects this parameter ID, it will copy the value into the parameter value register.
   // It will then trigger the next rung to read the next parameter of data.
   // The timer is a delay to give system enough time to copy the value into the register.
   64: XIC(rd_raw_var.1)[MOV(16#49B1,Out_hi6200.Parameter_ID) ,EQU(Inp_hi6200.Parameter_ID,16#49B1) COP(Inp_hi6200.Parameter_Value,pm_49B1,1) TON(read_delay_20,?,?) ];
   // Once timer is done, will clear bit for previous rung and turn on bit to run next rung.
   65: XIC(read_delay_20.DN)OTU(rd_raw_var.1)OTL(rd_raw_var.2);
   // The rung will set a parameter ID into the output table.  Once the input table reflects this parameter ID, it will copy the value into the parameter value register.
   // It will then trigger the next rung to read the next parameter of data.
   // The timer is a delay to give system enough time to copy the value into the register.
   66: XIC(rd_raw_var.2)[MOV(16#49B2,Out_hi6200.Parameter_ID) ,EQU(Inp_hi6200.Parameter_ID,16#49B2) COP(Inp_hi6200.Parameter_Value,pm_49B2,1) TON(read_delay_21,?,?) ];
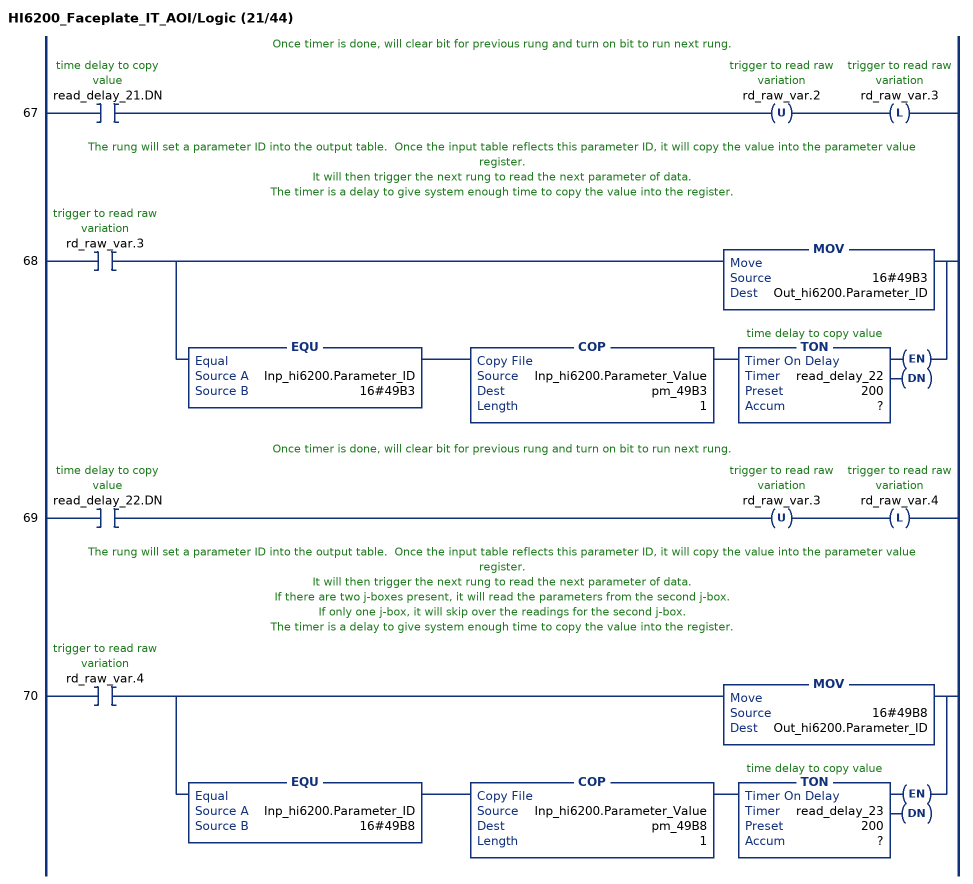
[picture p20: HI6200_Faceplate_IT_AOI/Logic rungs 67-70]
   // Once timer is done, will clear bit for previous rung and turn on bit to run next rung.
   67: XIC(read_delay_21.DN)OTU(rd_raw_var.2)OTL(rd_raw_var.3);
   // The rung will set a parameter ID into the output table.  Once the input table reflects this parameter ID, it will copy the value into the parameter value register.
   // It will then trigger the next rung to read the next parameter of data.
   // The timer is a delay to give system enough time to copy the value into the register.
   68: XIC(rd_raw_var.3)[MOV(16#49B3,Out_hi6200.Parameter_ID) ,EQU(Inp_hi6200.Parameter_ID,16#49B3) COP(Inp_hi6200.Parameter_Value,pm_49B3,1) TON(read_delay_22,?,?) ];
   // Once timer is done, will clear bit for previous rung and turn on bit to run next rung.
   69: XIC(read_delay_22.DN)OTU(rd_raw_var.3)OTL(rd_raw_var.4);
   // The rung will set a parameter ID into the output table.  Once the input table reflects this parameter ID, it will copy the value into the parameter value register.
   // It will then trigger the next rung to read the next parameter of data.
   // If there are two j-boxes present, it will read the parameters from the second j-box.
   // If only one j-box, it will skip over the readings for the second j-box.
   // The timer is a delay to give system enough time to copy the value into the register.
   70: XIC(rd_raw_var.4)[MOV(16#49B8,Out_hi6200.Parameter_ID) ,EQU(Inp_hi6200.Parameter_ID,16#49B8) COP(Inp_hi6200.Parameter_Value,pm_49B8,1) TON(read_delay_23,?,?) ];
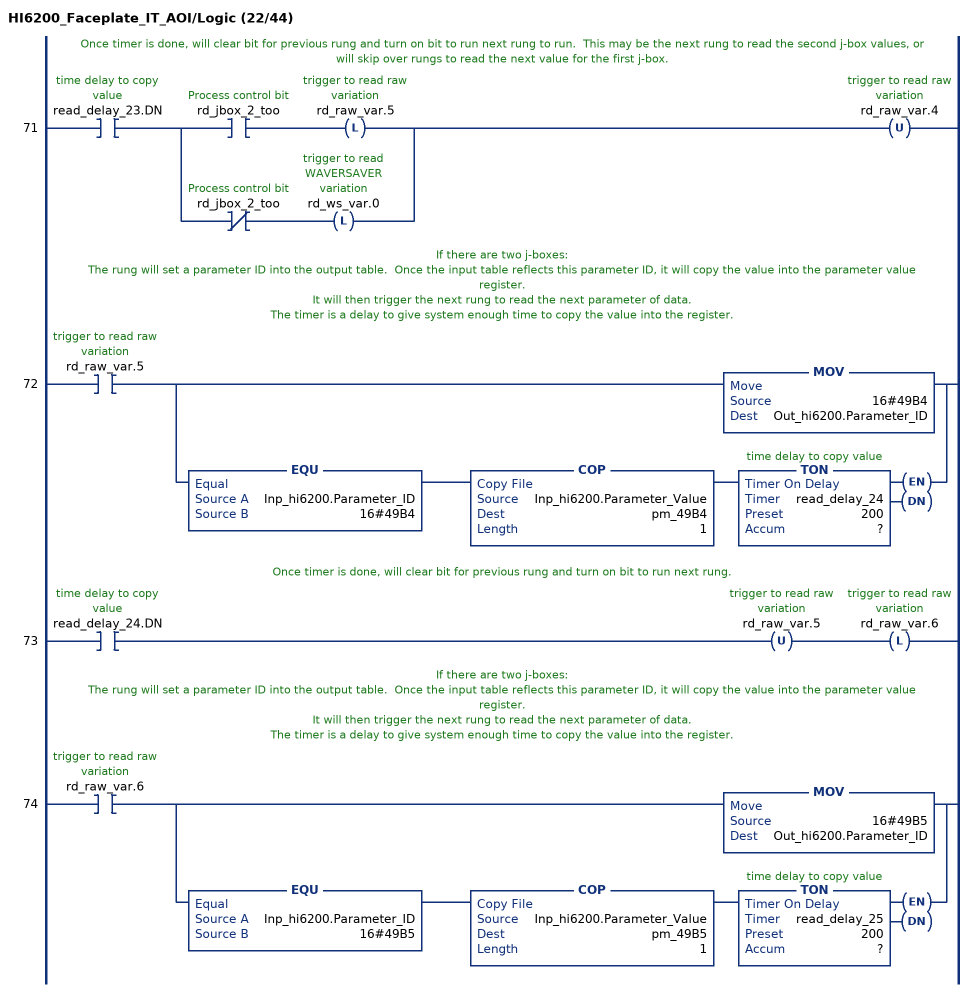
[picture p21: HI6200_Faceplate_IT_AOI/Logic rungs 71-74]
   // Once timer is done, will clear bit for previous rung and turn on bit to run next rung to run.  This may be the next rung to read the second j-box values, or will skip over rungs to read the next value for the first j-box.
   71: XIC(read_delay_23.DN)[XIC(rd_jbox_2_too) OTL(rd_raw_var.5) ,XIO(rd_jbox_2_too) OTL(rd_ws_var.0) ]OTU(rd_raw_var.4);
   // If there are two j-boxes:
   // The rung will set a parameter ID into the output table.  Once the input table reflects this parameter ID, it will copy the value into the parameter value register.
   // It will then trigger the next rung to read the next parameter of data.
   // The timer is a delay to give system enough time to copy the value into the register.
   72: XIC(rd_raw_var.5)[MOV(16#49B4,Out_hi6200.Parameter_ID) ,EQU(Inp_hi6200.Parameter_ID,16#49B4) COP(Inp_hi6200.Parameter_Value,pm_49B4,1) TON(read_delay_24,?,?) ];
   // Once timer is done, will clear bit for previous rung and turn on bit to run next rung.
   73: XIC(read_delay_24.DN)OTU(rd_raw_var.5)OTL(rd_raw_var.6);
   // If there are two j-boxes:
   // The rung will set a parameter ID into the output table.  Once the input table reflects this parameter ID, it will copy the value into the parameter value register.
   // It will then trigger the next rung to read the next parameter of data.
   // The timer is a delay to give system enough time to copy the value into the register.
   74: XIC(rd_raw_var.6)[MOV(16#49B5,Out_hi6200.Parameter_ID) ,EQU(Inp_hi6200.Parameter_ID,16#49B5) COP(Inp_hi6200.Parameter_Value,pm_49B5,1) TON(read_delay_25,?,?) ];
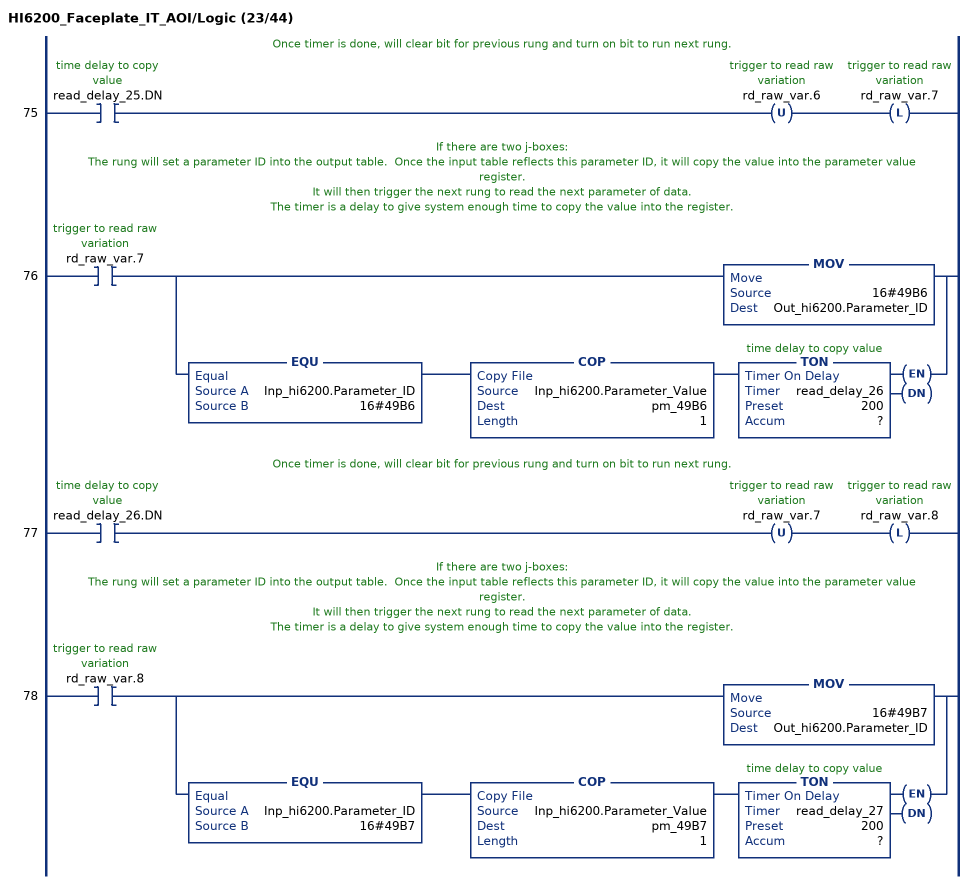
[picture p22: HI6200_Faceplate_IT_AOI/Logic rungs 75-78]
   // Once timer is done, will clear bit for previous rung and turn on bit to run next rung.
   75: XIC(read_delay_25.DN)OTU(rd_raw_var.6)OTL(rd_raw_var.7);
   // If there are two j-boxes:
   // The rung will set a parameter ID into the output table.  Once the input table reflects this parameter ID, it will copy the value into the parameter value register.
   // It will then trigger the next rung to read the next parameter of data.
   // The timer is a delay to give system enough time to copy the value into the register.
   76: XIC(rd_raw_var.7)[MOV(16#49B6,Out_hi6200.Parameter_ID) ,EQU(Inp_hi6200.Parameter_ID,16#49B6) COP(Inp_hi6200.Parameter_Value,pm_49B6,1) TON(read_delay_26,?,?) ];
   // Once timer is done, will clear bit for previous rung and turn on bit to run next rung.
   77: XIC(read_delay_26.DN)OTU(rd_raw_var.7)OTL(rd_raw_var.8);
   // If there are two j-boxes:
   // The rung will set a parameter ID into the output table.  Once the input table reflects this parameter ID, it will copy the value into the parameter value register.
   // It will then trigger the next rung to read the next parameter of data.
   // The timer is a delay to give system enough time to copy the value into the register.
   78: XIC(rd_raw_var.8)[MOV(16#49B7,Out_hi6200.Parameter_ID) ,EQU(Inp_hi6200.Parameter_ID,16#49B7) COP(Inp_hi6200.Parameter_Value,pm_49B7,1) TON(read_delay_27,?,?) ];
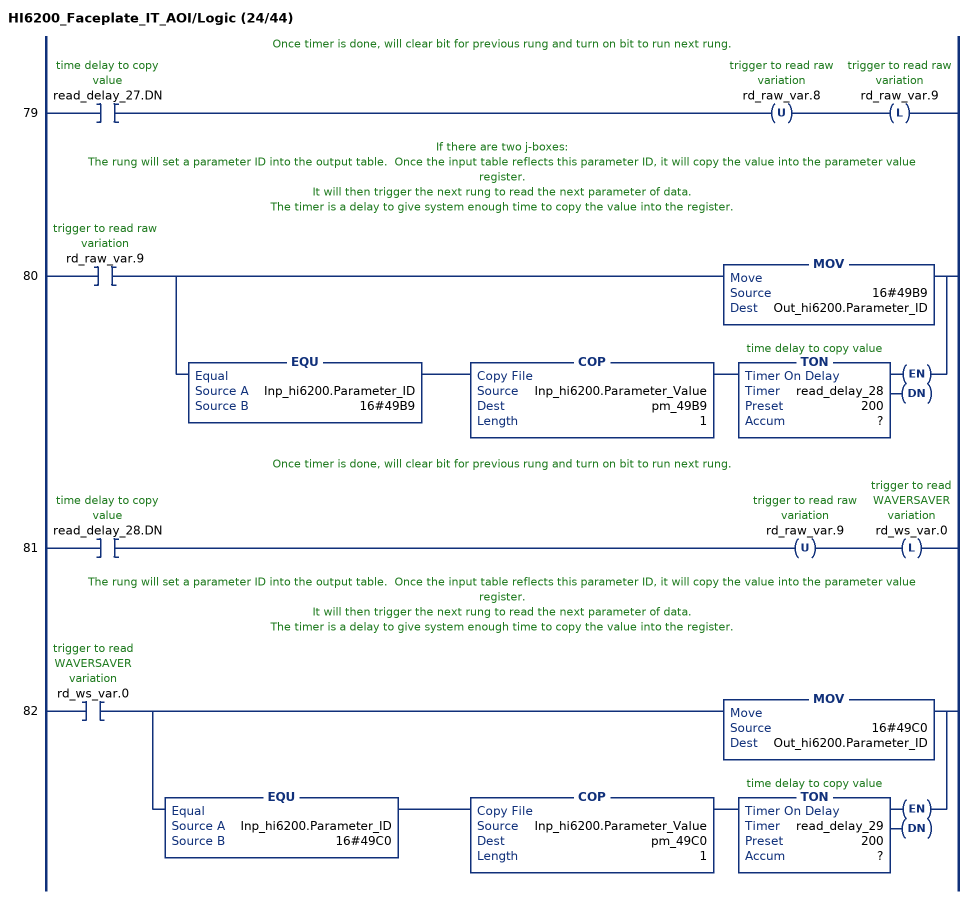
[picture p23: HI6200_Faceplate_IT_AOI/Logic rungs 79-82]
   // Once timer is done, will clear bit for previous rung and turn on bit to run next rung.
   79: XIC(read_delay_27.DN)OTU(rd_raw_var.8)OTL(rd_raw_var.9);
   // If there are two j-boxes:
   // The rung will set a parameter ID into the output table.  Once the input table reflects this parameter ID, it will copy the value into the parameter value register.
   // It will then trigger the next rung to read the next parameter of data.
   // The timer is a delay to give system enough time to copy the value into the register.
   80: XIC(rd_raw_var.9)[MOV(16#49B9,Out_hi6200.Parameter_ID) ,EQU(Inp_hi6200.Parameter_ID,16#49B9) COP(Inp_hi6200.Parameter_Value,pm_49B9,1) TON(read_delay_28,?,?) ];
   // Once timer is done, will clear bit for previous rung and turn on bit to run next rung.
   81: XIC(read_delay_28.DN)OTU(rd_raw_var.9)OTL(rd_ws_var.0);
   // The rung will set a parameter ID into the output table.  Once the input table reflects this parameter ID, it will copy the value into the parameter value register.
   // It will then trigger the next rung to read the next parameter of data.
   // The timer is a delay to give system enough time to copy the value into the register.
   82: XIC(rd_ws_var.0)[MOV(16#49C0,Out_hi6200.Parameter_ID) ,EQU(Inp_hi6200.Parameter_ID,16#49C0) COP(Inp_hi6200.Parameter_Value,pm_49C0,1) TON(read_delay_29,?,?) ];
